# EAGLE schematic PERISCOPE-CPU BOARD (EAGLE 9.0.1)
This Set of Many Schematics Is what comprises the Revision-A PCB, of my eden project "PERISCOPE".

## Sheet 1 of 14: Clock, Horizontal Sync
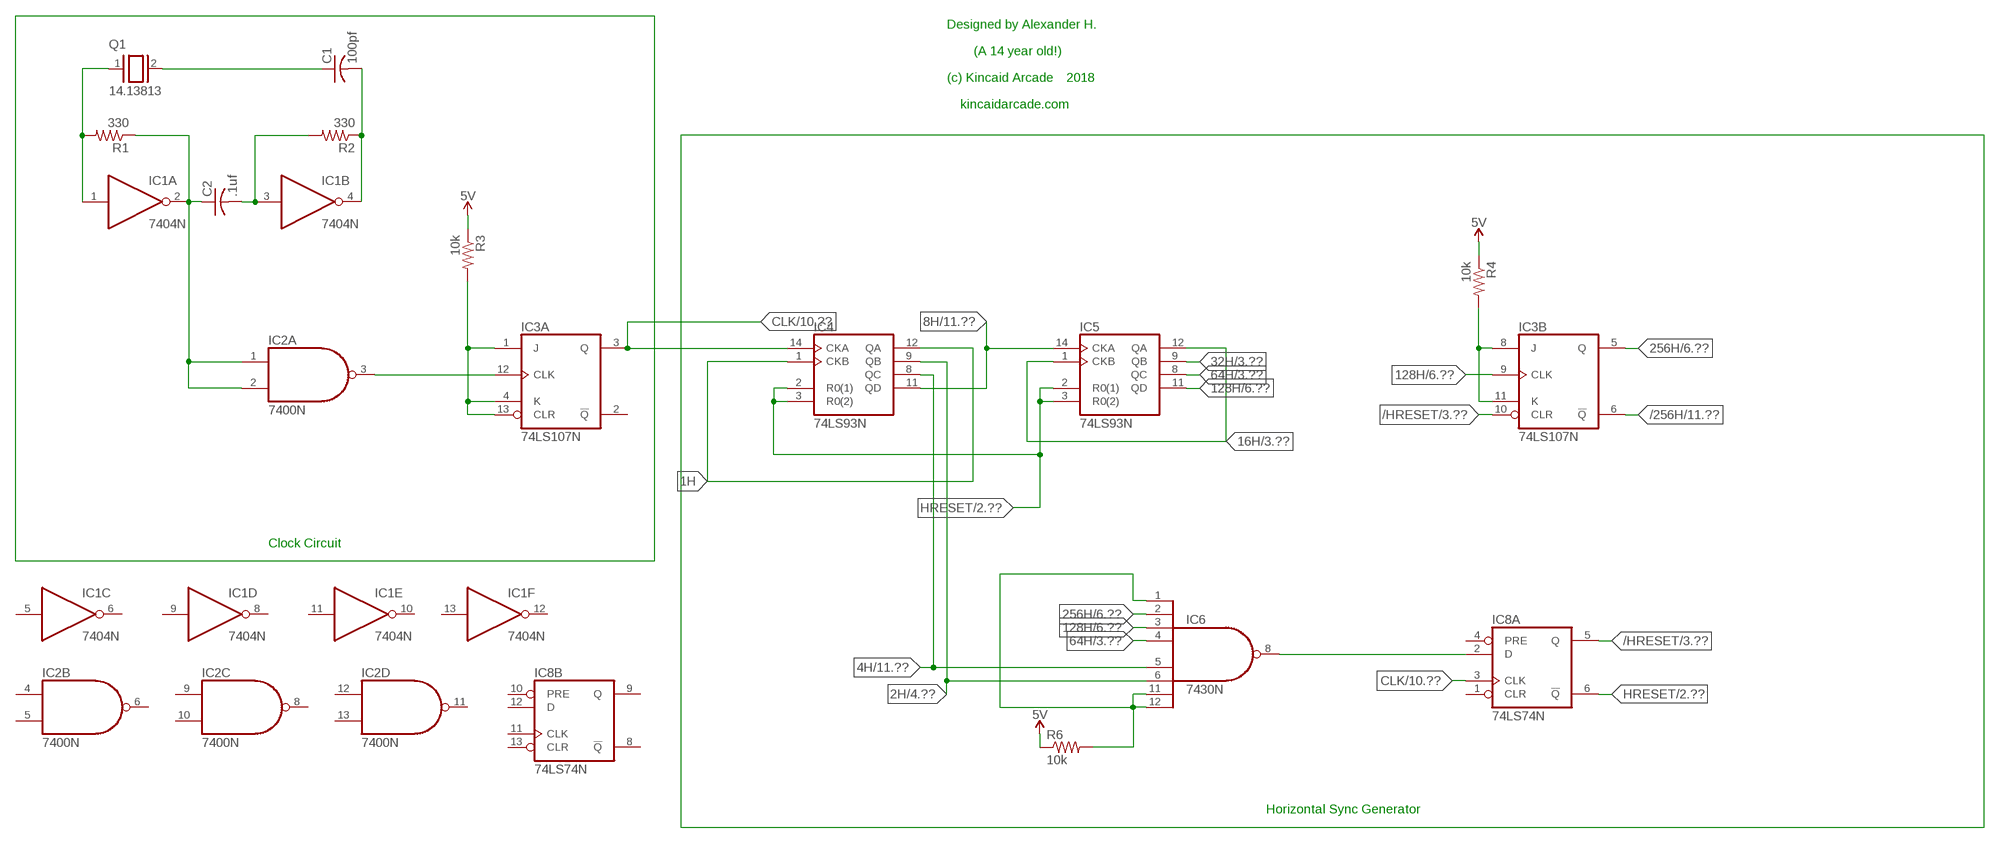
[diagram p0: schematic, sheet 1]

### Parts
C1  100pf  C-US050-025X075  [C050-025X075]
C2  .1uf  C-US050-025X075  [C050-025X075]
IC1  7404N  [DIL14]
IC2  7400N  [DIL14]
IC3  74LS107N  [DIL14]
IC4  74LS93N  [DIL14]
IC5  74LS93N  [DIL14]
IC6  7430N  [DIL14]
IC8  74LS74N  [DIL14]
Q1  14.13813  XTAL/S  [QS]
R1  330  R-US_0207/10  [0207/10]
R2  330  R-US_0207/10  [0207/10]
R3  10k  R-US_0207/10  [0207/10]
R4  10k  R-US_0207/10  [0207/10]
R6  10k  R-US_0207/10  [0207/10]

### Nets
1H: IC4.1(CKB) IC4.12(QA)
2H: IC4.9(QB) IC6.6(I5) ; also sheet 4
4H: IC4.8(QC) IC6.5(I4) ; also sheet 11
5V: R3.1 R4.1 R6.1 ; also sheet 2
8H: IC4.11(QD) IC5.14(CKA) ; also sheet 11
16H: IC5.1(CKB) IC5.12(QA) ; also sheet 3,6,11
32H: IC5.9(QB) ; also sheet 3,6,11
64H: IC5.8(QC) IC6.4(I3) ; also sheet 3,6,11
128H: IC3.9(B:CLK) IC5.11(QD) IC6.3(I2) ; also sheet 6,11
256H: IC3.5(B:Q) IC6.2(I1) ; also sheet 6,11
512H: IC6.1(I0) IC6.11(I6) IC6.12(I7) R6.2
/256H: IC3.6(B:!Q) ; also sheet 11
/HRESET: IC3.10(B:CLR) IC8.5(A:Q) ; also sheet 3
CLK: IC3.3(A:Q) IC4.14(CKA) IC8.3(A:CLK) ; also sheet 10
HRESET: IC4.2(R0(1)) IC4.3(R0(2)) IC5.2(R0(1)) IC5.3(R0(2)) IC8.6(A:!Q) ; also sheet 2,7,8,10
N$1: C1.1 Q1.2
N$2: C1.2 IC1.4(B:O) R2.1
N$3: C2.1 IC1.2(A:O) IC2.1(A:I0) IC2.2(A:I1) R1.1
N$4: C2.2 IC1.3(B:I) R2.2
N$5: IC1.1(A:I) Q1.1 R1.2
N$6: IC2.3(A:O) IC3.12(A:CLK)
N$7: IC3.1(A:J) IC3.4(A:K) IC3.13(A:CLR) R3.2
N$8: IC3.8(B:J) IC3.11(B:K) R4.2
N$11: IC6.8(O) IC8.2(A:D)
Unconnected: IC1.5(C:I) IC1.6(C:O) IC1.8(D:O) IC1.9(D:I) IC1.10(E:O) IC1.11(E:I) IC1.12(F:O) IC1.13(F:I) IC2.4(B:I0) IC2.5(B:I1) IC2.6(B:O) IC2.8(C:O) IC2.9(C:I0) IC2.10(C:I1) IC2.11(D:O) IC2.12(D:I0) IC2.13(D:I1) IC3.2(A:!Q) IC8.1(A:CLR) IC8.4(A:PRE) IC8.8(B:!Q) IC8.9(B:Q) IC8.10(B:PRE) IC8.11(B:CLK) IC8.12(B:D) IC8.13(B:CLR)

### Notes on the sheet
- Designed by Alexander H.
- (A 14 year old!)
- (c) Kincaid Arcade | 2018
- kincaidarcade.com
- Clock Circuit
- Horizontal Sync Generator

## Sheet 2 of 14: Vertical Sync Generator
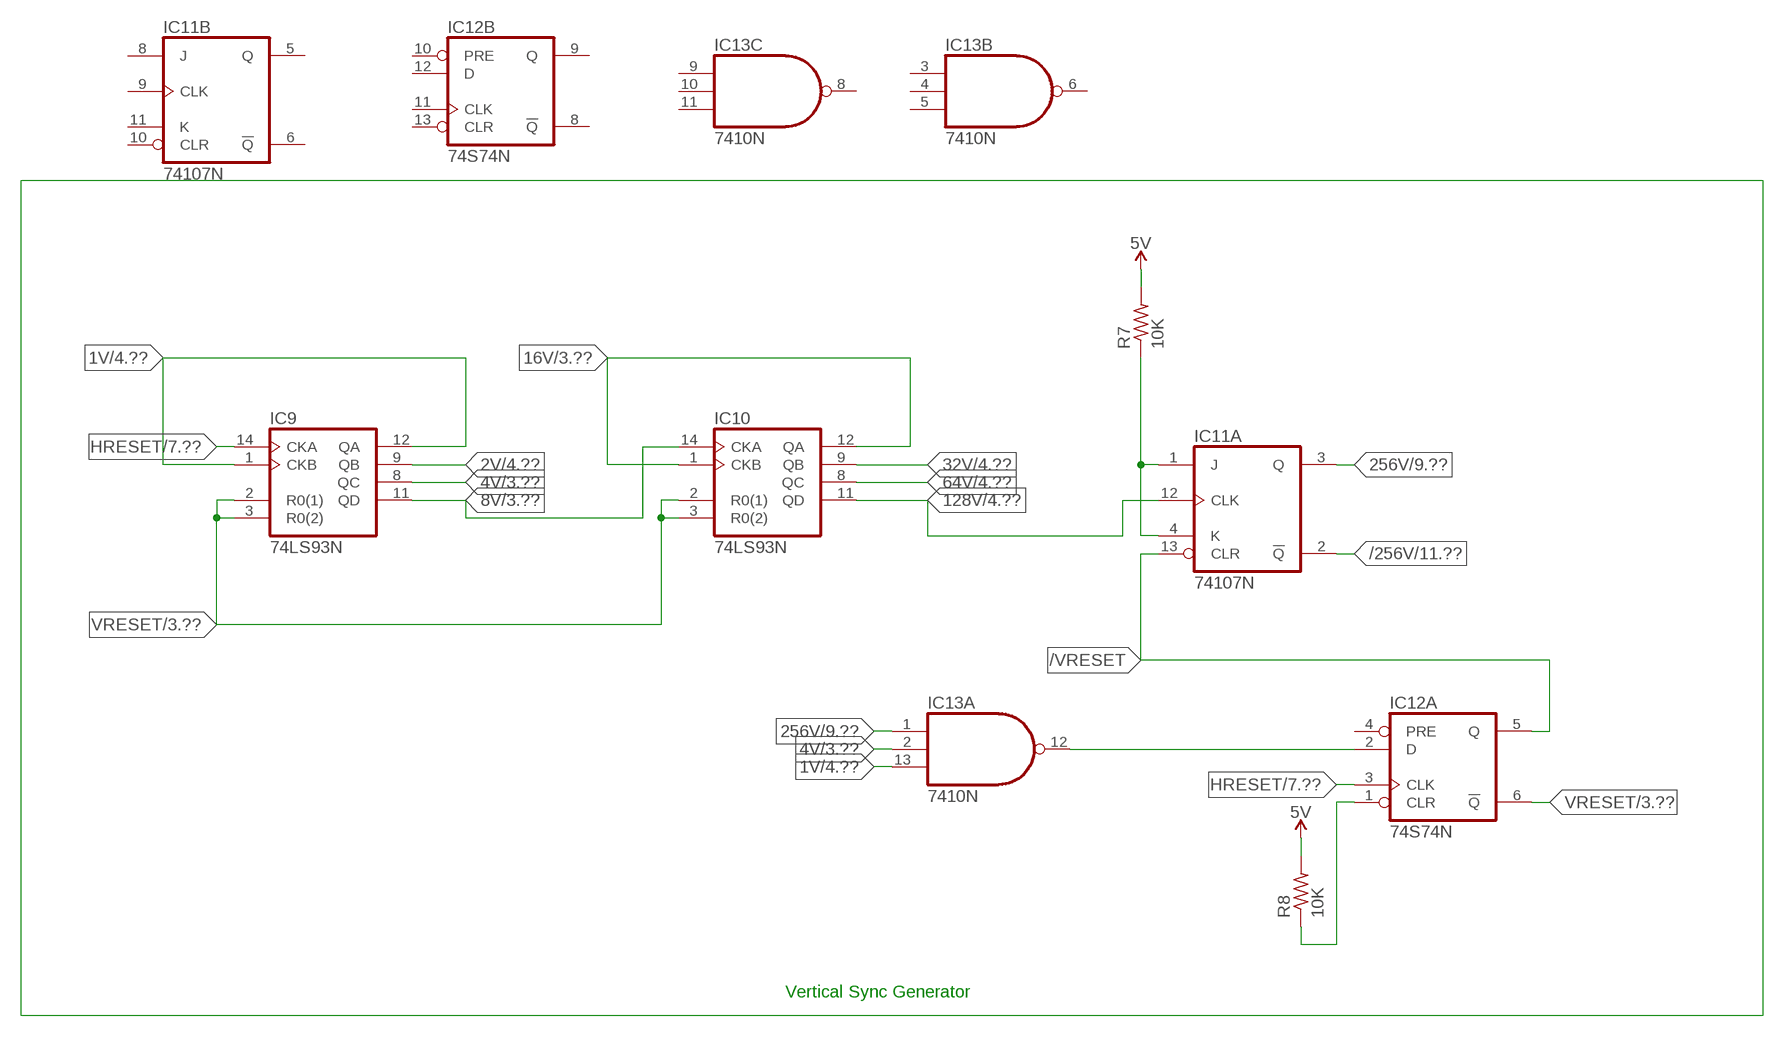
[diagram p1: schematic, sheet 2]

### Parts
IC9  74LS93N  [DIL14]
IC10  74LS93N  [DIL14]
IC11  74107N  [DIL14]
IC12  74S74N  [DIL14]
IC13  7410N  [DIL14]
R7  10K  R-US_0207/10  [0207/10]
R8  10K  R-US_0207/10  [0207/10]

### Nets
1V: IC9.1(CKB) IC9.12(QA) IC13.13(A:I2) ; also sheet 4
2V: IC9.9(QB) ; also sheet 4
4V: IC9.8(QC) IC13.2(A:I1) ; also sheet 3,4,11
5V: R7.2 R8.2 ; also sheet 1
8V: IC9.11(QD) IC10.14(CKA) ; also sheet 3,4,11
16V: IC10.1(CKB) IC10.12(QA) ; also sheet 3,4,5,11
32V: IC10.9(QB) ; also sheet 4,5,11
64V: IC10.8(QC) ; also sheet 4,5
128V: IC10.11(QD) IC11.12(A:CLK) ; also sheet 4,5,9,11
256V: IC11.3(A:Q) IC13.1(A:I0) ; also sheet 9
/256V: IC11.2(A:!Q) ; also sheet 11
/VRESET: IC11.13(A:CLR) IC12.5(A:Q)
HRESET: IC9.14(CKA) IC12.3(A:CLK) ; also sheet 1,7,8,10
N$15: IC11.1(A:J) IC11.4(A:K) R7.1
N$16: IC12.1(A:CLR) R8.1
N$17: IC12.2(A:D) IC13.12(A:O)
VRESET: IC9.2(R0(1)) IC9.3(R0(2)) IC10.2(R0(1)) IC10.3(R0(2)) IC12.6(A:!Q) ; also sheet 3,5
Unconnected: IC11.5(B:Q) IC11.6(B:!Q) IC11.8(B:J) IC11.9(B:CLK) IC11.10(B:CLR) IC11.11(B:K) IC12.4(A:PRE) IC12.8(B:!Q) IC12.9(B:Q) IC12.10(B:PRE) IC12.11(B:CLK) IC12.12(B:D) IC12.13(B:CLR) IC13.3(B:I0) IC13.4(B:I1) IC13.5(B:I2) IC13.6(B:O) IC13.8(C:O) IC13.9(C:I0) IC13.10(C:I1) IC13.11(C:I2)

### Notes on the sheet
- Vertical Sync Generator

## Sheet 3 of 14: Sync Generation
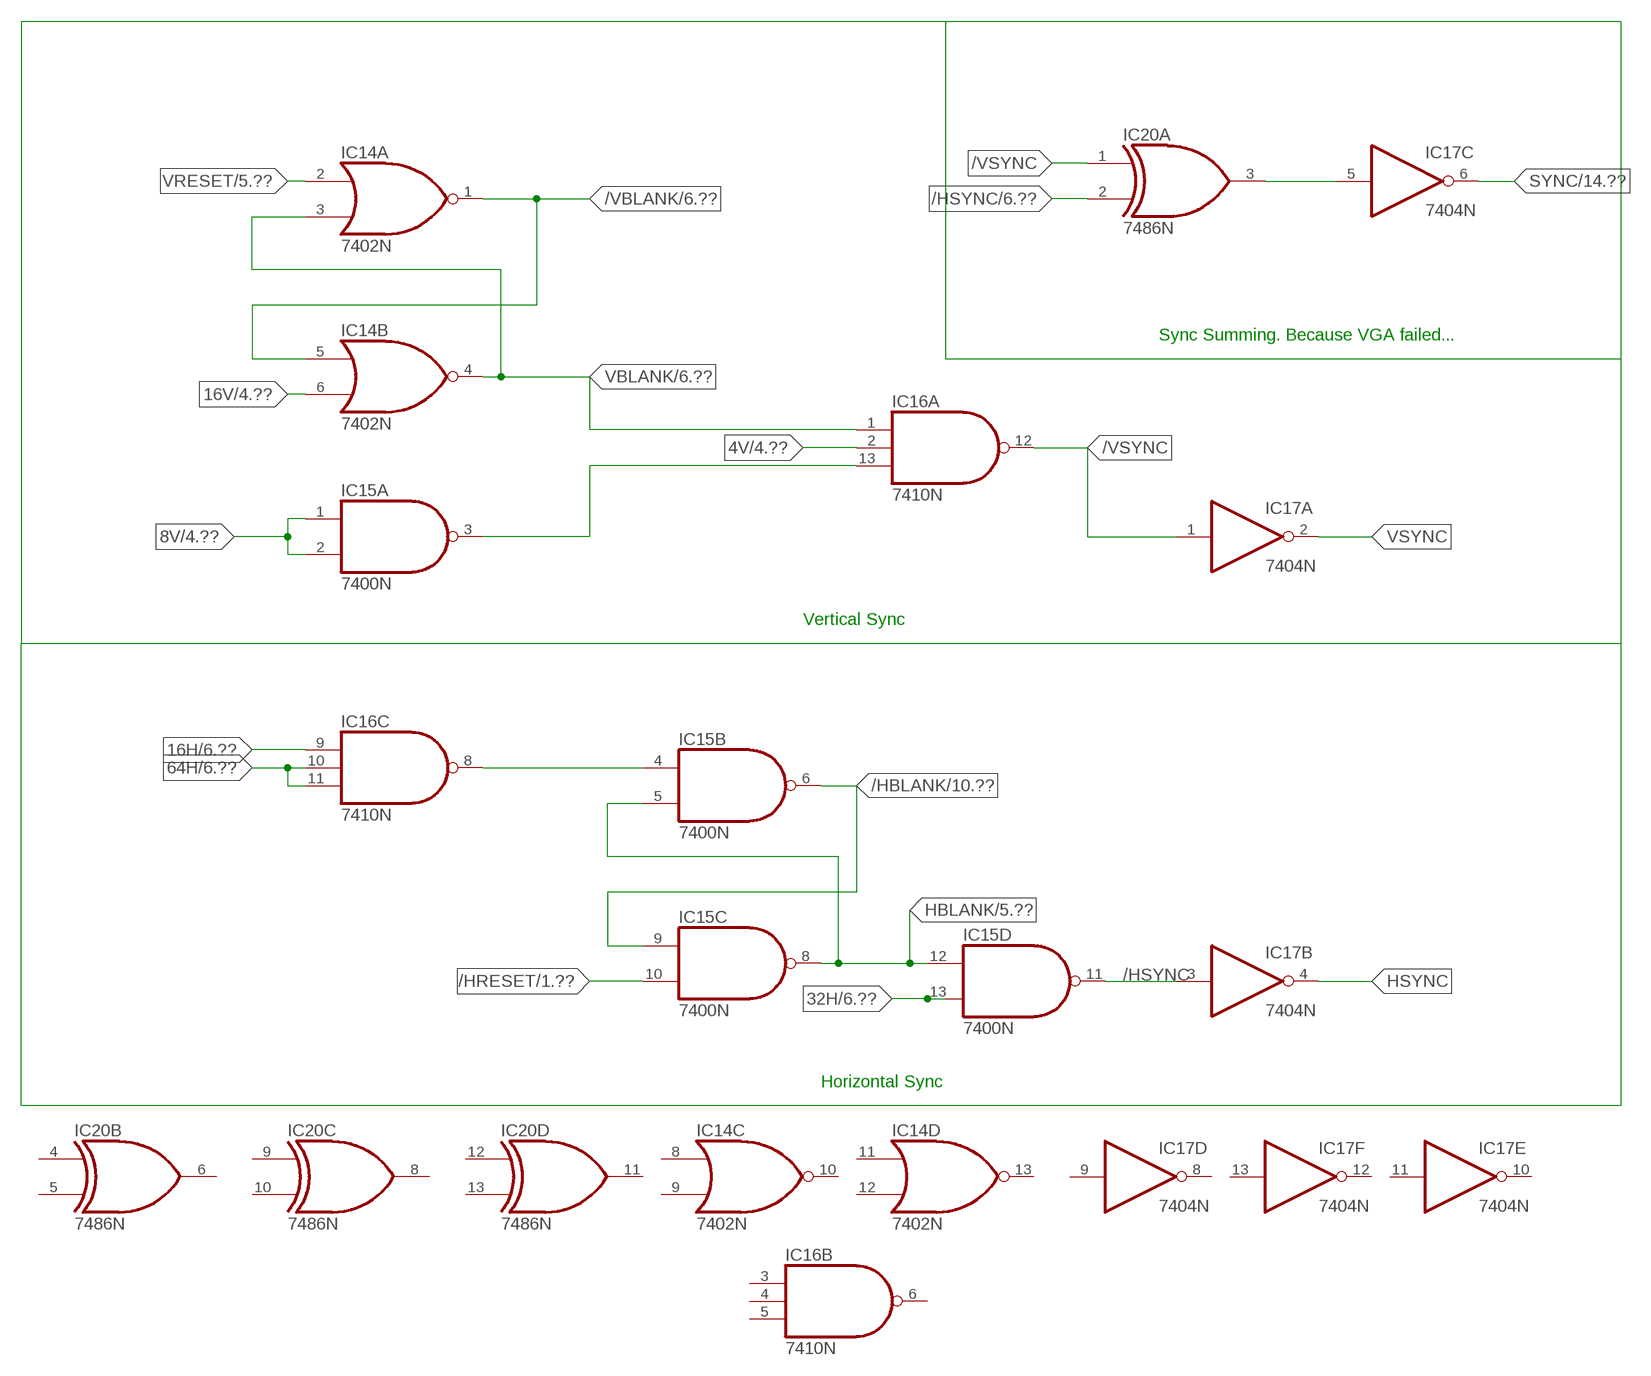
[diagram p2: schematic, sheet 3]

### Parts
IC14  7402N  [DIL14]
IC15  7400N  [DIL14]
IC16  7410N  [DIL14]
IC17  7404N  [DIL14]
IC20  7486N  [DIL14]

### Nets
4V: IC16.2(A:I1) ; also sheet 2,4,11
8V: IC15.1(A:I0) IC15.2(A:I1) ; also sheet 2,4,11
16H: IC16.9(C:I0) ; also sheet 1,6,11
16V: IC14.6(B:I1) ; also sheet 2,4,5,11
32H: IC15.13(D:I1) ; also sheet 1,6,11
64H: IC16.10(C:I1) IC16.11(C:I2) ; also sheet 1,6,11
/HBLANK: IC15.6(B:O) IC15.9(C:I0) ; also sheet 10
/HRESET: IC15.10(C:I1) ; also sheet 1
/HSYNC: IC15.11(D:O) IC17.3(B:I) IC20.2(A:I1) ; also sheet 6,10
/VBLANK: IC14.1(A:O) IC14.5(B:I0) ; also sheet 6,10
/VSYNC: IC16.12(A:O) IC17.1(A:I) IC20.1(A:I0)
HBLANK: IC15.5(B:I1) IC15.8(C:O) IC15.12(D:I0) ; also sheet 5,10
HSYNC: IC17.4(B:O)
N$19: IC15.4(B:I0) IC16.8(C:O)
N$20: IC15.3(A:O) IC16.13(A:I2)
N$22: IC17.5(C:I) IC20.3(A:O)
SYNC: IC17.6(C:O) ; also sheet 14
VBLANK: IC14.3(A:I1) IC14.4(B:O) IC16.1(A:I0) ; also sheet 6
VRESET: IC14.2(A:I0) ; also sheet 2,5
VSYNC: IC17.2(A:O)
Unconnected: IC14.8(C:I0) IC14.9(C:I1) IC14.10(C:O) IC14.11(D:I0) IC14.12(D:I1) IC14.13(D:O) IC16.3(B:I0) IC16.4(B:I1) IC16.5(B:I2) IC16.6(B:O) IC17.8(D:O) IC17.9(D:I) IC17.10(E:O) IC17.11(E:I) IC17.12(F:O) IC17.13(F:I) IC20.4(B:I0) IC20.5(B:I1) IC20.6(B:O) IC20.8(C:O) IC20.9(C:I0) IC20.10(C:I1) IC20.11(D:O) IC20.12(D:I0) IC20.13(D:I1)

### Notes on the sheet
- Sync Summing. Because VGA failed...
- Vertical Sync
- Horizontal Sync

## Sheet 4 of 14: Ocean Generation, Surface and Floor
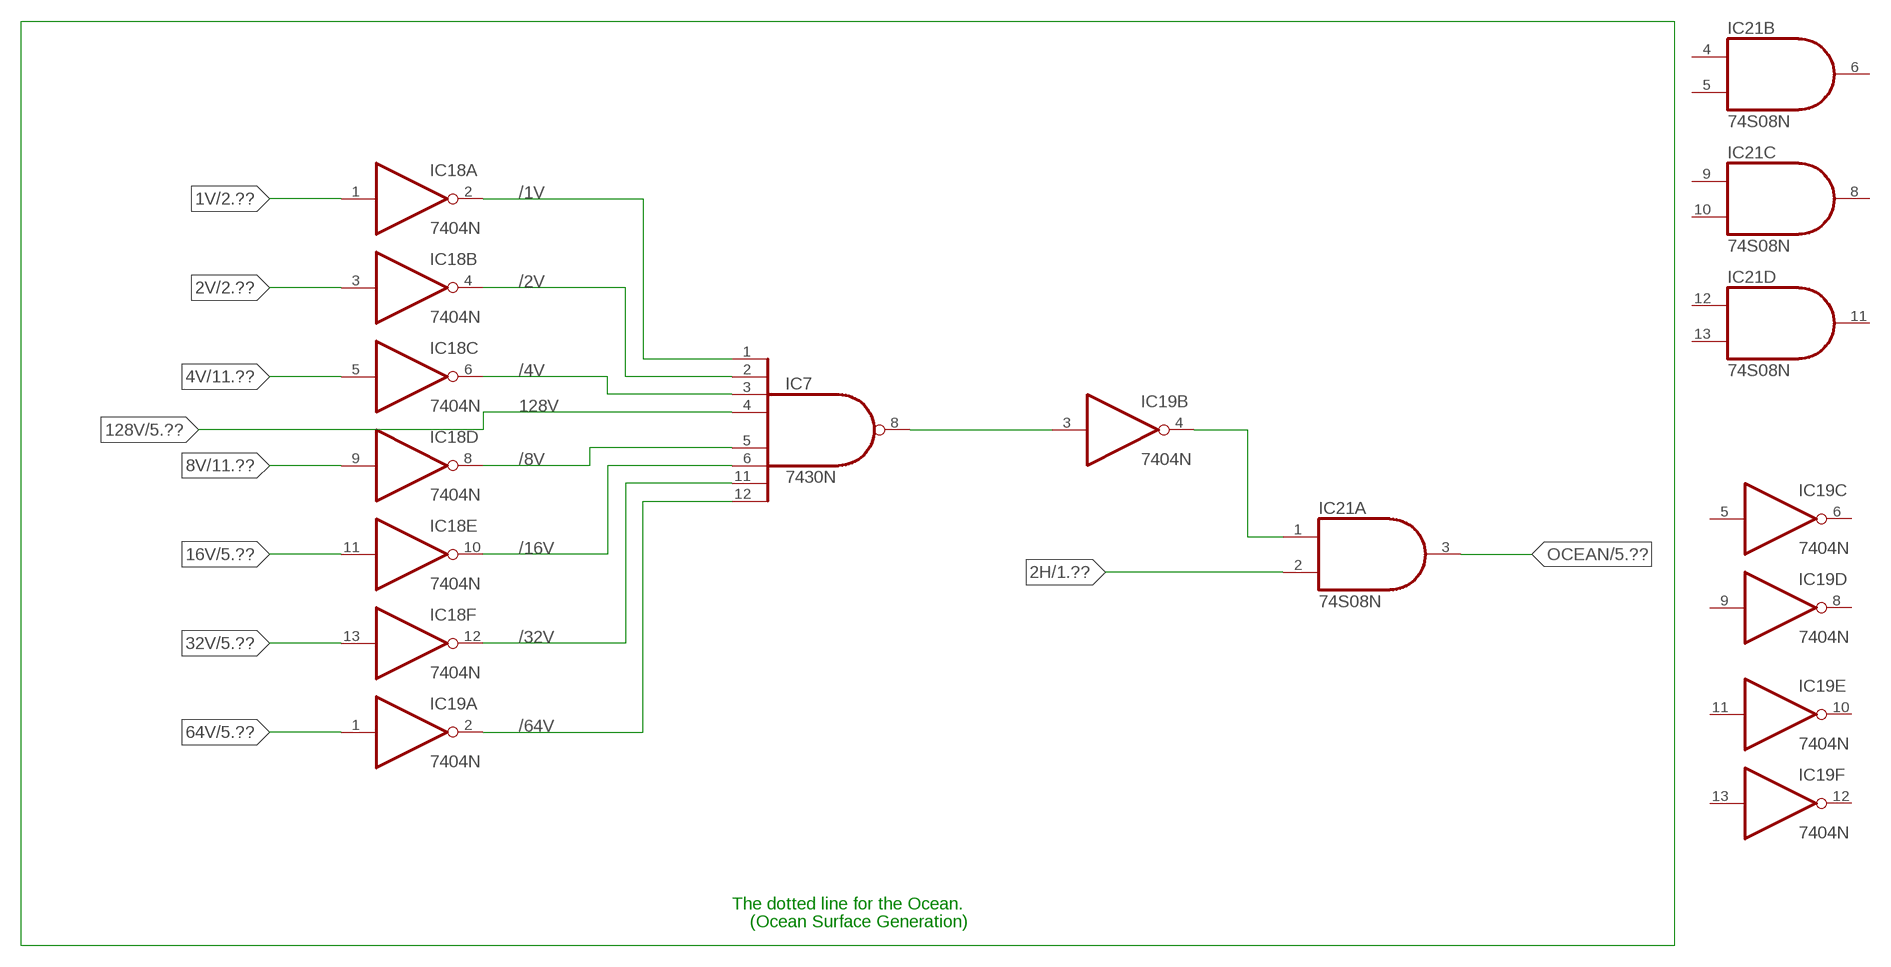
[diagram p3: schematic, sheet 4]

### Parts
IC7  7430N  [DIL14]
IC18  7404N  [DIL14]
IC19  7404N  [DIL14]
IC21  74S08N  [DIL14]

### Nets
1V: IC18.1(A:I) ; also sheet 2
2H: IC21.2(A:I1) ; also sheet 1
2V: IC18.3(B:I) ; also sheet 2
4V: IC18.5(C:I) ; also sheet 2,3,11
8V: IC18.9(D:I) ; also sheet 2,3,11
16V: IC18.11(E:I) ; also sheet 2,3,5,11
32V: IC18.13(F:I) ; also sheet 2,5,11
64V: IC19.1(A:I) ; also sheet 2,5
128V: IC7.4(I3) ; also sheet 2,5,9,11
/1V: IC7.1(I0) IC18.2(A:O)
/2V: IC7.2(I1) IC18.4(B:O)
/4V: IC7.3(I2) IC18.6(C:O)
/8V: IC7.5(I4) IC18.8(D:O)
/16V: IC7.6(I5) IC18.10(E:O)
/32V: IC7.11(I6) IC18.12(F:O)
/64V: IC7.12(I7) IC19.2(A:O) ; also sheet 11
N$28: IC7.8(O) IC19.3(B:I)
N$29: IC19.4(B:O) IC21.1(A:I0)
OCEAN: IC21.3(A:O) ; also sheet 5,6,10,13
Unconnected: IC19.5(C:I) IC19.6(C:O) IC19.8(D:O) IC19.9(D:I) IC19.10(E:O) IC19.11(E:I) IC19.12(F:O) IC19.13(F:I) IC21.4(B:I0) IC21.5(B:I1) IC21.6(B:O) IC21.8(C:O) IC21.9(C:I0) IC21.10(C:I1) IC21.11(D:O) IC21.12(D:I0) IC21.13(D:I1)

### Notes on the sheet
- The dotted line for the Ocean.
- (Ocean Surface Generation)

## Sheet 5 of 14: Freighter Generation
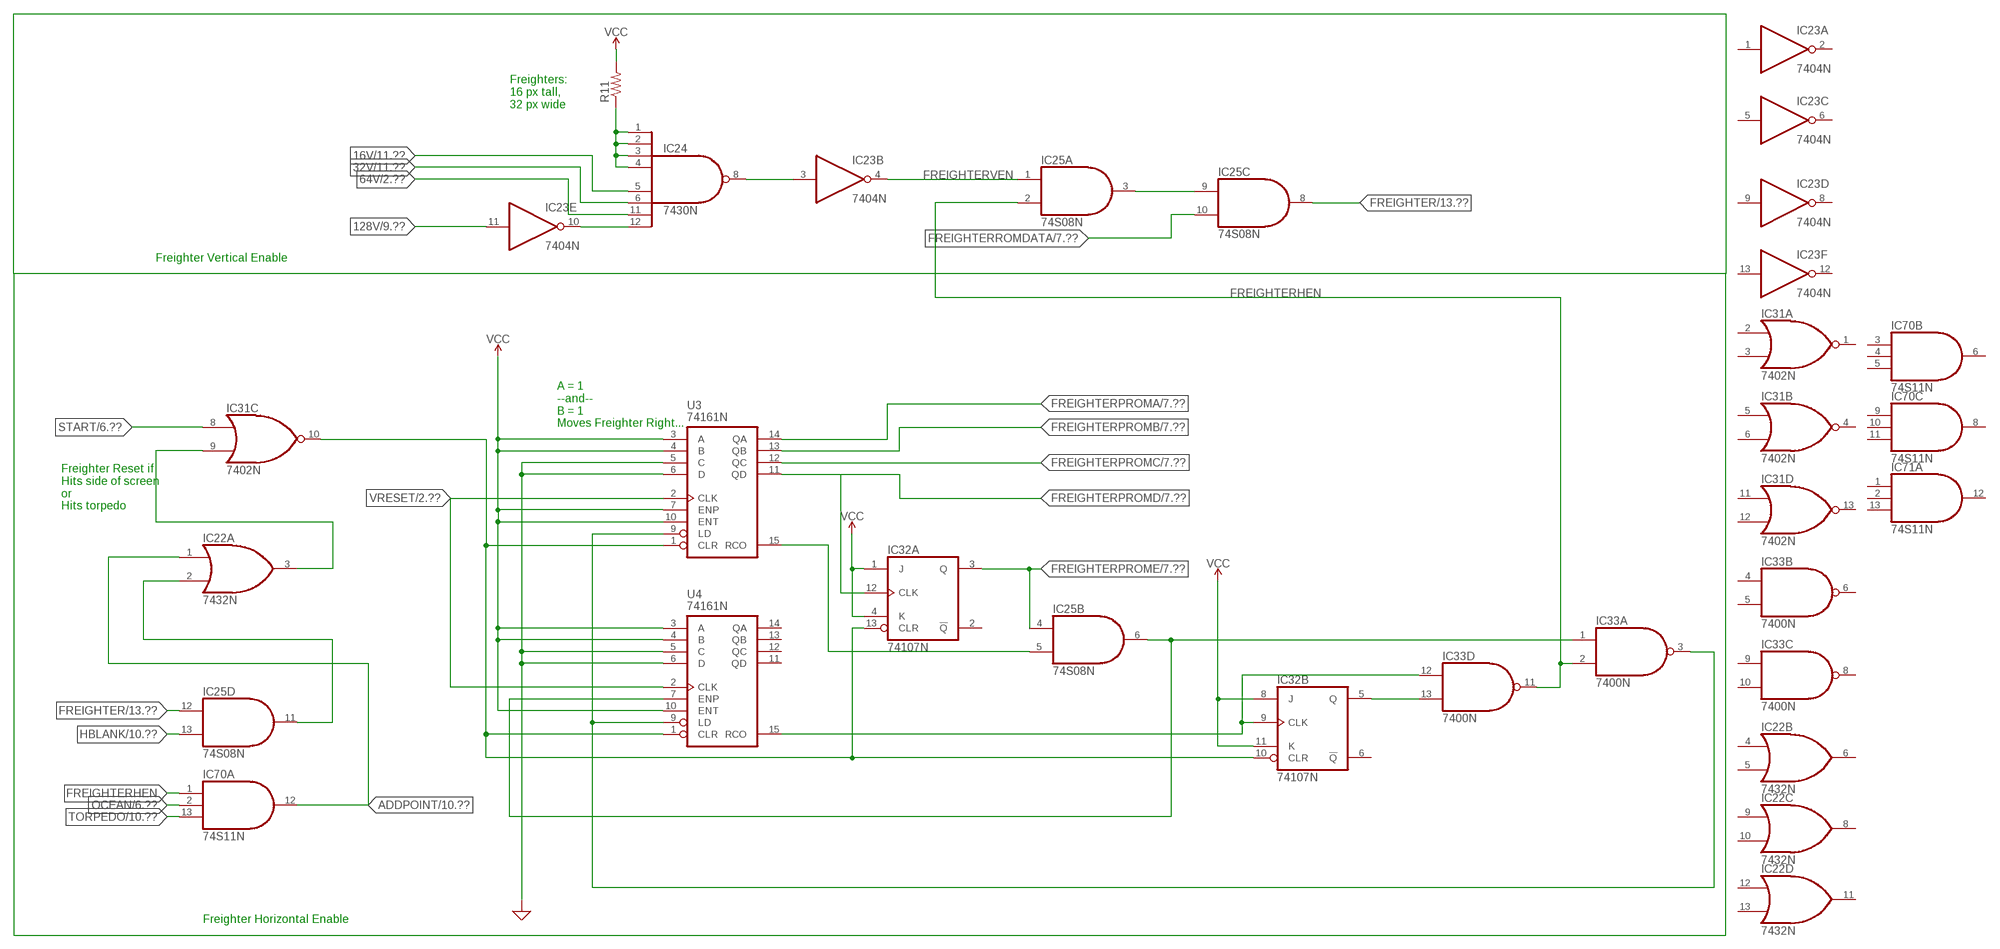
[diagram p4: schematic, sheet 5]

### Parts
IC22  7432N  [DIL14]
IC23  7404N  [DIL14]
IC24  7430N  [DIL14]
IC25  74S08N  [DIL14]
IC31  7402N  [DIL14]
IC32  74107N  [DIL14]
IC33  7400N  [DIL14]
IC70  74S11N  [DIL14]
IC71  74S11N  [DIL14]
R11  R-US_0207/10  [0207/10]
U3  74161N  [DIL16]
U4  74161N  [DIL16]

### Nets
16V: IC24.5(I4) ; also sheet 2,3,4,11
32V: IC24.6(I5) ; also sheet 2,4,11
64V: IC24.11(I6) ; also sheet 2,4
128V: IC23.11(E:I) ; also sheet 2,4,9,11
ADDPOINT: IC22.1(A:I0) IC70.12(A:O) ; also sheet 10,11
FREIGHTER: IC25.8(C:O) IC25.12(D:I0) ; also sheet 13
FREIGHTERHEN: IC25.2(A:I1) IC33.2(A:I1) IC33.11(D:O) IC70.1(A:I0)
FREIGHTERPROMA: U3.14(QA) ; also sheet 7
FREIGHTERPROMB: U3.13(QB) ; also sheet 7
FREIGHTERPROMC: U3.12(QC) ; also sheet 7
FREIGHTERPROMD: IC32.12(A:CLK) U3.11(QD) ; also sheet 7
FREIGHTERPROME: IC25.4(B:I0) IC32.3(A:Q) ; also sheet 7
FREIGHTERROMDATA: IC25.10(C:I1) ; also sheet 7
FREIGHTERVEN: IC23.4(B:O) IC25.1(A:I0) ; also sheet 7
GND: U3.5(C) U3.6(D) U4.5(C) U4.6(D) ; supply symbol labelled SUP ; also sheet 6,7,8,9,10,11,14
HBLANK: IC22.3(A:O) IC25.13(D:I1) IC31.9(C:I1) ; also sheet 3,10
N$21: IC31.10(C:O) IC32.10(B:CLR) IC32.13(A:CLR) U3.1(CLR) U4.1(CLR)
N$24: IC25.5(B:I1) U3.15(RCO)
N$25: IC25.6(B:O) IC33.1(A:I0) U4.7(ENP)
N$27: IC32.5(B:Q) IC33.13(D:I1)
N$31: IC22.2(A:I1) IC25.11(D:O)
N$35: IC23.10(E:O) IC24.12(I7)
N$36: IC23.3(B:I) IC24.8(O)
N$37: IC25.3(A:O) IC25.9(C:I0)
N$40: IC24.1(I0) IC24.2(I1) IC24.3(I2) IC24.4(I3) R11.1
N$53: IC32.9(B:CLK) IC33.12(D:I0) U4.15(RCO)
N$54: IC33.3(A:O) U3.9(LD) U4.9(LD)
OCEAN: IC70.2(A:I1) ; also sheet 4,6,10,13
START: IC31.8(C:I0) ; also sheet 6,9,11
TORPEDO: IC70.13(A:I2) ; also sheet 10,13
VCC: IC32.1(A:J) IC32.4(A:K) IC32.8(B:J) IC32.11(B:K) R11.2 U3.3(A) U3.4(B) U3.7(ENP) U3.10(ENT) U4.3(A) U4.4(B) U4.10(ENT) ; also sheet 6,7,8,9,10,11,14
VRESET: U3.2(CLK) U4.2(CLK) ; also sheet 2,3
Unconnected: IC22.4(B:I0) IC22.5(B:I1) IC22.6(B:O) IC22.8(C:O) IC22.9(C:I0) IC22.10(C:I1) IC22.11(D:O) IC22.12(D:I0) IC22.13(D:I1) IC23.1(A:I) IC23.2(A:O) IC23.5(C:I) IC23.6(C:O) IC23.8(D:O) IC23.9(D:I) IC23.12(F:O) IC23.13(F:I) IC31.1(A:O) IC31.2(A:I0) IC31.3(A:I1) IC31.4(B:O) IC31.5(B:I0) IC31.6(B:I1) IC31.11(D:I0) IC31.12(D:I1) IC31.13(D:O) IC32.2(A:!Q) IC32.6(B:!Q) IC33.4(B:I0) IC33.5(B:I1) IC33.6(B:O) IC33.8(C:O) IC33.9(C:I0) IC33.10(C:I1) IC70.3(B:I0) IC70.4(B:I1) IC70.5(B:I2) IC70.6(B:O) IC70.8(C:O) IC70.9(C:I0) IC70.10(C:I1) IC70.11(C:I2) IC71.1(A:I0) IC71.2(A:I1) IC71.3(B:I0) IC71.4(B:I1) IC71.5(B:I2) IC71.6(B:O) IC71.8(C:O) IC71.9(C:I0) IC71.10(C:I1) IC71.11(C:I2) IC71.12(A:O) IC71.13(A:I2) U4.11(QD) U4.12(QC) U4.13(QB) U4.14(QA)

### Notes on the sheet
- Freighters:
  16 px tall,
  32 px wide
- Freighter Vertical Enable
- A = 1 
  --and--
  B = 1
  Moves Freighter Right...
- Freighter Reset if 
  Hits side of screen
  or
  Hits torpedo
- Freighter Horizontal Enable

## Sheet 6 of 14: Submarine Generation
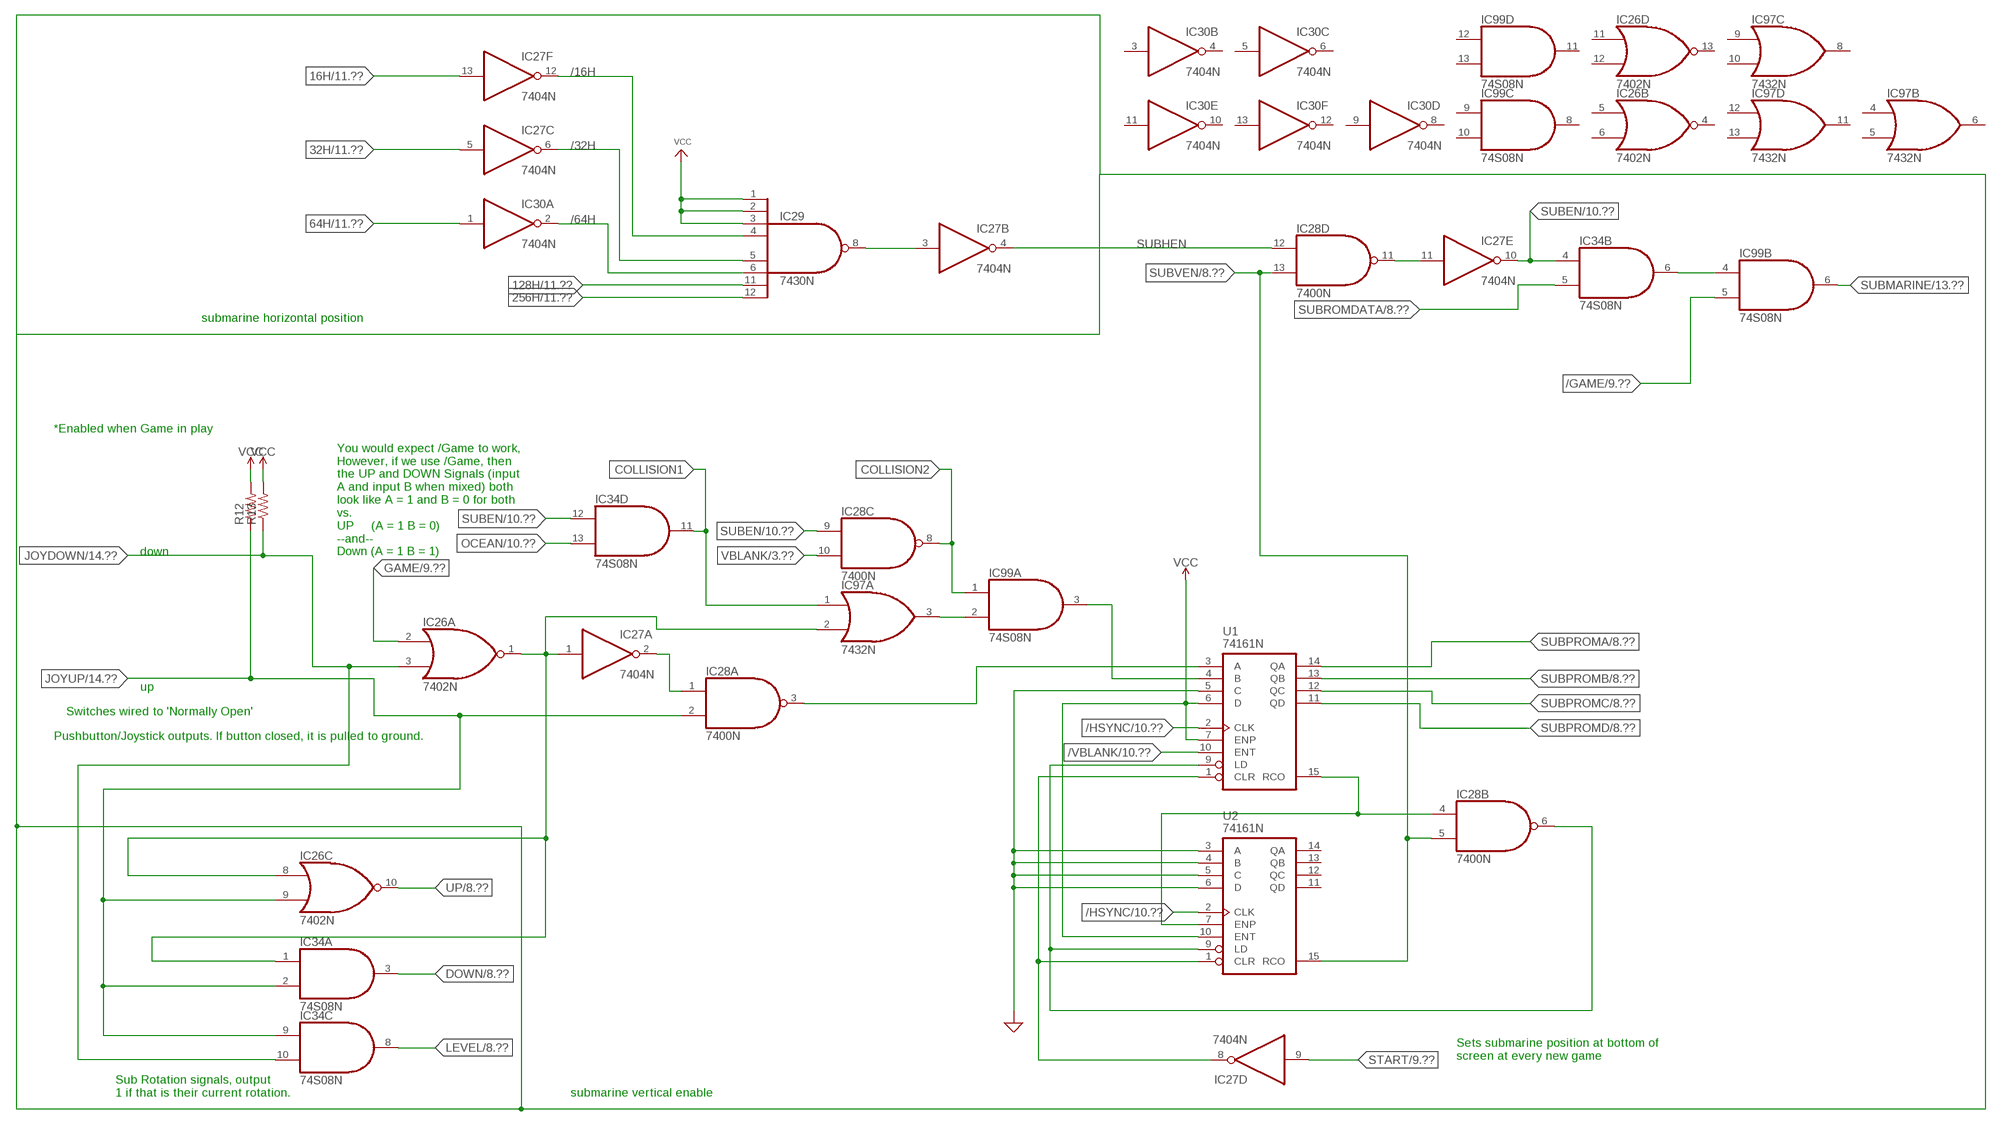
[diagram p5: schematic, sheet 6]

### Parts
IC26  7402N  [DIL14]
IC27  7404N  [DIL14]
IC28  7400N  [DIL14]
IC29  7430N  [DIL14]
IC30  7404N  [DIL14]
IC34  74S08N  [DIL14]
IC97  7432N  [DIL14]
IC99  74S08N  [DIL14]
R12  R-US_0207/10  [0207/10]
R13  R-US_0207/10  [0207/10]
U1  74161N  [DIL16]
U2  74161N  [DIL16]

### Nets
16H: IC27.13(F:I) ; also sheet 1,3,11
32H: IC27.5(C:I) ; also sheet 1,3,11
64H: IC30.1(A:I) ; also sheet 1,3,11
128H: IC29.11(I6) ; also sheet 1,11
256H: IC29.12(I7) ; also sheet 1,11
/16H: IC27.12(F:O) IC29.4(I3)
/32H: IC27.6(C:O) IC29.5(I4) ; also sheet 11
/64H: IC29.6(I5) IC30.2(A:O) ; also sheet 11
/GAME: IC99.5(B:I1) ; also sheet 9,10
/HSYNC: U1.2(CLK) U2.2(CLK) ; also sheet 3,10
/VBLANK: U1.10(ENT) ; also sheet 3,10
COLLISION1: IC34.11(D:O) IC97.1(A:I0)
COLLISION2: IC28.8(C:O) IC99.1(A:I0)
DOWN: IC34.3(A:O) ; also sheet 8,10
GAME: IC26.2(A:I0) ; also sheet 9
GND: U1.5(C) U2.3(A) U2.4(B) U2.5(C) U2.6(D) ; supply symbol labelled SUP ; also sheet 5,7,8,9,10,11,14
GSTART: IC27.8(D:O) U1.1(CLR) U2.1(CLR)
JOYDOWN: IC26.3(A:I1) IC34.10(C:I1) R13.1 ; also sheet 14
JOYUP: IC26.9(C:I1) IC28.2(A:I1) IC34.2(A:I1) IC34.9(C:I0) R12.1 ; also sheet 14
LEVEL: IC34.8(C:O) ; also sheet 8
N$42: IC27.2(A:O) IC28.1(A:I0)
N$43: IC26.1(A:O) IC26.8(C:I0) IC27.1(A:I) IC34.1(A:I0) IC97.2(A:I1)
N$44: IC28.4(B:I0) U1.15(RCO) U2.7(ENP)
N$45: IC27.3(B:I) IC29.8(O)
N$46: IC28.6(B:O) U1.9(LD) U2.9(LD)
N$47: IC27.11(E:I) IC28.11(D:O)
N$48: IC97.3(A:O) IC99.2(A:I1)
N$186: IC99.3(A:O) U1.4(B)
N$190: IC28.3(A:O) U1.3(A)
N$210: IC34.6(B:O) IC99.4(B:I0)
OCEAN: IC34.13(D:I1) ; also sheet 4,5,10,13
START: IC27.9(D:I) ; also sheet 5,9,11
SUBEN: IC27.10(E:O) IC28.9(C:I0) IC34.4(B:I0) IC34.12(D:I0) ; also sheet 10
SUBHEN: IC27.4(B:O) IC28.12(D:I0) ; also sheet 10
SUBMARINE: IC99.6(B:O) ; also sheet 13
SUBPROMA: U1.14(QA) ; also sheet 8,10
SUBPROMB: U1.13(QB) ; also sheet 8,10
SUBPROMC: U1.12(QC) ; also sheet 8,10
SUBPROMD: U1.11(QD) ; also sheet 8,10
SUBROMDATA: IC34.5(B:I1) ; also sheet 8
SUBVEN: IC28.5(B:I1) IC28.13(D:I1) U2.15(RCO) ; also sheet 8,10
UP: IC26.10(C:O) ; also sheet 8,10
VBLANK: IC28.10(C:I1) ; also sheet 3
VCC: IC29.1(I0) IC29.2(I1) IC29.3(I2) R12.2 R13.2 U1.6(D) U1.7(ENP) U2.10(ENT) ; also sheet 5,7,8,9,10,11,14
Unconnected: IC26.4(B:O) IC26.5(B:I0) IC26.6(B:I1) IC26.11(D:I0) IC26.12(D:I1) IC26.13(D:O) IC30.3(B:I) IC30.4(B:O) IC30.5(C:I) IC30.6(C:O) IC30.8(D:O) IC30.9(D:I) IC30.10(E:O) IC30.11(E:I) IC30.12(F:O) IC30.13(F:I) IC97.4(B:I0) IC97.5(B:I1) IC97.6(B:O) IC97.8(C:O) IC97.9(C:I0) IC97.10(C:I1) IC97.11(D:O) IC97.12(D:I0) IC97.13(D:I1) IC99.8(C:O) IC99.9(C:I0) IC99.10(C:I1) IC99.11(D:O) IC99.12(D:I0) IC99.13(D:I1) U2.11(QD) U2.12(QC) U2.13(QB) U2.14(QA)

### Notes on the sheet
- submarine horizontal position
- *Enabled when Game in play
- down
- You would expect /Game to work,
  However, if we use /Game, then 
  the UP and DOWN Signals (input
  A and input B when mixed) both
  look like A = 1 and B = 0 for both
  vs. 
  UP     (A = 1 B = 0)
  --and--
  Down (A = 1 B = 1)
- up
- Switches wired to 'Normally Open'
- Pushbutton/Joystick outputs. If button closed, it is pulled to ground.
- Sets submarine position at bottom of
  screen at every new game
- Sub Rotation signals, output
  1 if that is their current rotation.
- submarine vertical enable

## Sheet 7 of 14: Freighter Prom data/addressing
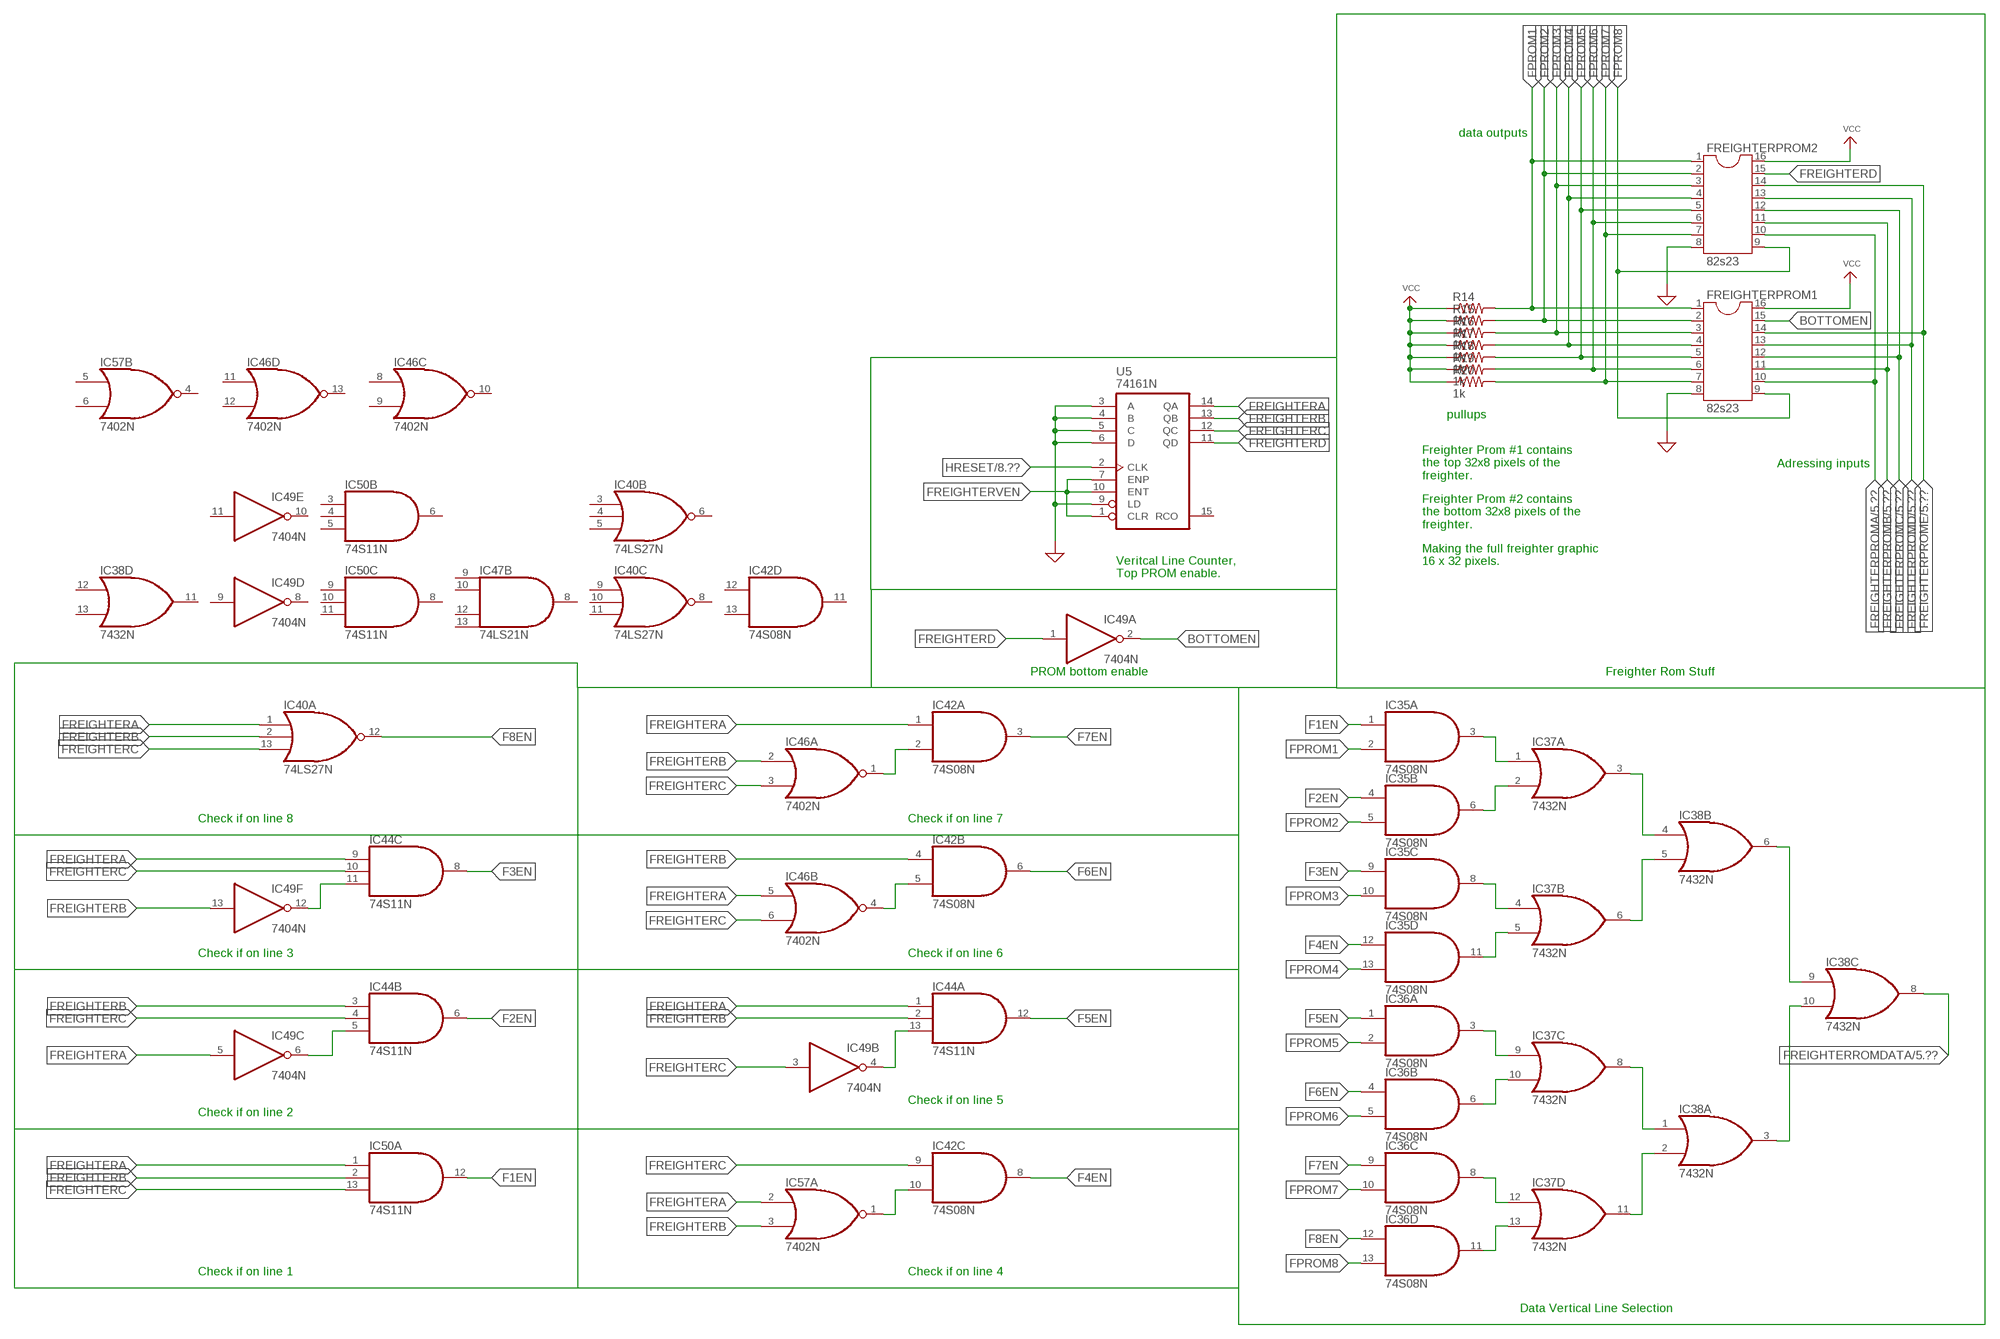
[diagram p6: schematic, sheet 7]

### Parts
FREIGHTERPROM1  82s23  DIL16  [DIL16]
FREIGHTERPROM2  82s23  DIL16  [DIL16]
IC35  74S08N  [DIL14]
IC36  74S08N  [DIL14]
IC37  7432N  [DIL14]
IC38  7432N  [DIL14]
IC40  74LS27N  [DIL14]
IC42  74S08N  [DIL14]
IC44  74S11N  [DIL14]
IC46  7402N  [DIL14]
IC47  74LS21N  [DIL14]
IC49  7404N  [DIL14]
IC50  74S11N  [DIL14]
IC57  7402N  [DIL14]
R14  1k  R-US_0207/10  [0207/10]
R15  1k  R-US_0207/10  [0207/10]
R16  1k  R-US_0207/10  [0207/10]
R17  1k  R-US_0207/10  [0207/10]
R18  1k  R-US_0207/10  [0207/10]
R19  1k  R-US_0207/10  [0207/10]
R20  1k  R-US_0207/10  [0207/10]
U5  74161N  [DIL16]

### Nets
BOTTOMEN: FREIGHTERPROM1.15 IC49.2(A:O)
F1EN: IC35.1(A:I0) IC50.12(A:O)
F2EN: IC35.4(B:I0) IC44.6(B:O)
F3EN: IC35.9(C:I0) IC44.8(C:O)
F4EN: IC35.12(D:I0) IC42.8(C:O)
F5EN: IC36.1(A:I0) IC44.12(A:O)
F6EN: IC36.4(B:I0) IC42.6(B:O)
F7EN: IC36.9(C:I0) IC42.3(A:O)
F8EN: IC36.12(D:I0) IC40.12(A:O)
FPROM1: FREIGHTERPROM1.1 FREIGHTERPROM2.1 IC35.2(A:I1) R14.2
FPROM2: FREIGHTERPROM1.2 FREIGHTERPROM2.2 IC35.5(B:I1) R15.2
FPROM3: FREIGHTERPROM1.3 FREIGHTERPROM2.3 IC35.10(C:I1) R16.2
FPROM4: FREIGHTERPROM1.4 FREIGHTERPROM2.4 IC35.13(D:I1) R17.2
FPROM5: FREIGHTERPROM1.5 FREIGHTERPROM2.5 IC36.2(A:I1) R18.2
FPROM6: FREIGHTERPROM1.6 FREIGHTERPROM2.6 IC36.5(B:I1) R19.2
FPROM7: FREIGHTERPROM1.7 FREIGHTERPROM2.7 IC36.10(C:I1) R20.2
FPROM8: FREIGHTERPROM1.9 FREIGHTERPROM2.9 IC36.13(D:I1)
FREIGHTERA: IC40.1(A:I0) IC42.1(A:I0) IC44.1(A:I0) IC44.9(C:I0) IC46.5(B:I0) IC49.5(C:I) IC50.1(A:I0) IC57.2(A:I0) U5.14(QA)
FREIGHTERB: IC40.2(A:I1) IC42.4(B:I0) IC44.2(A:I1) IC44.3(B:I0) IC46.2(A:I0) IC49.13(F:I) IC50.2(A:I1) IC57.3(A:I1) U5.13(QB)
FREIGHTERC: IC40.13(A:I2) IC42.9(C:I0) IC44.4(B:I1) IC44.10(C:I1) IC46.3(A:I1) IC46.6(B:I1) IC49.3(B:I) IC50.13(A:I2) U5.12(QC)
FREIGHTERD: FREIGHTERPROM2.15 IC49.1(A:I) U5.11(QD)
FREIGHTERPROMA: FREIGHTERPROM1.10 FREIGHTERPROM2.10 ; also sheet 5
FREIGHTERPROMB: FREIGHTERPROM1.11 FREIGHTERPROM2.11 ; also sheet 5
FREIGHTERPROMC: FREIGHTERPROM1.12 FREIGHTERPROM2.12 ; also sheet 5
FREIGHTERPROMD: FREIGHTERPROM1.13 FREIGHTERPROM2.13 ; also sheet 5
FREIGHTERPROME: FREIGHTERPROM1.14 FREIGHTERPROM2.14 ; also sheet 5
FREIGHTERROMDATA: IC38.8(C:O) ; also sheet 5
FREIGHTERVEN: U5.1(CLR) U5.7(ENP) U5.10(ENT) ; also sheet 5
GND: FREIGHTERPROM1.8 FREIGHTERPROM2.8 U5.3(A) U5.4(B) U5.5(C) U5.6(D) U5.9(LD) ; supply symbol labelled SUP ; also sheet 5,6,8,9,10,11,14
HRESET: U5.2(CLK) ; also sheet 1,2,8,10
N$41: IC35.6(B:O) IC37.2(A:I1)
N$51: IC35.3(A:O) IC37.1(A:I0)
N$52: IC35.8(C:O) IC37.4(B:I0)
N$55: IC35.11(D:O) IC37.5(B:I1)
N$56: IC36.3(A:O) IC37.9(C:I0)
N$57: IC36.6(B:O) IC37.10(C:I1)
N$58: IC36.8(C:O) IC37.12(D:I0)
N$59: IC36.11(D:O) IC37.13(D:I1)
N$60: IC37.11(D:O) IC38.2(A:I1)
N$61: IC37.8(C:O) IC38.1(A:I0)
N$62: IC37.6(B:O) IC38.5(B:I1)
N$63: IC37.3(A:O) IC38.4(B:I0)
N$64: IC38.6(B:O) IC38.9(C:I0)
N$65: IC38.3(A:O) IC38.10(C:I1)
N$66: IC42.10(C:I1) IC57.1(A:O)
N$67: IC44.13(A:I2) IC49.4(B:O)
N$69: IC42.5(B:I1) IC46.4(B:O)
N$70: IC42.2(A:I1) IC46.1(A:O)
N$72: IC44.5(B:I2) IC49.6(C:O)
N$73: IC44.11(C:I2) IC49.12(F:O)
VCC: FREIGHTERPROM1.16 FREIGHTERPROM2.16 R14.1 R15.1 R16.1 R17.1 R18.1 R19.1 R20.1 ; also sheet 5,6,8,9,10,11,14
Unconnected: IC38.11(D:O) IC38.12(D:I0) IC38.13(D:I1) IC40.3(B:I0) IC40.4(B:I1) IC40.5(B:I2) IC40.6(B:O) IC40.8(C:O) IC40.9(C:I0) IC40.10(C:I1) IC40.11(C:I2) IC42.11(D:O) IC42.12(D:I0) IC42.13(D:I1) IC46.8(C:I0) IC46.9(C:I1) IC46.10(C:O) IC46.11(D:I0) IC46.12(D:I1) IC46.13(D:O) IC47.1(A:I0) IC47.2(A:I1) IC47.4(A:I2) IC47.5(A:I3) IC47.6(A:O) IC47.8(B:O) IC47.9(B:I0) IC47.10(B:I1) IC47.12(B:I2) IC47.13(B:I3) IC49.8(D:O) IC49.9(D:I) IC49.10(E:O) IC49.11(E:I) IC50.3(B:I0) IC50.4(B:I1) IC50.5(B:I2) IC50.6(B:O) IC50.8(C:O) IC50.9(C:I0) IC50.10(C:I1) IC50.11(C:I2) IC57.4(B:O) IC57.5(B:I0) IC57.6(B:I1) IC57.8(C:I0) IC57.9(C:I1) IC57.10(C:O) IC57.11(D:I0) IC57.12(D:I1) IC57.13(D:O) U5.15(RCO)

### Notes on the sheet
- data outputs
- pullups
- Adressing inputs
- Freighter Prom #1 contains
  the top 32x8 pixels of the 
  freighter.
- Freighter Prom #2 contains
  the bottom 32x8 pixels of the 
  freighter.
- Making the full freighter graphic 
  16 x 32 pixels.
- Veritcal Line Counter,
  Top PROM enable.
- PROM bottom enable | Freighter Rom Stuff
- Check if on line 8 | Check if on line 7
- Check if on line 3 | Check if on line 6
- Check if on line 5
- Check if on line 2
- Check if on line 1 | Check if on line 4
- Data Vertical Line Selection

## Sheet 8 of 14: Submarine PROM data/addressing.
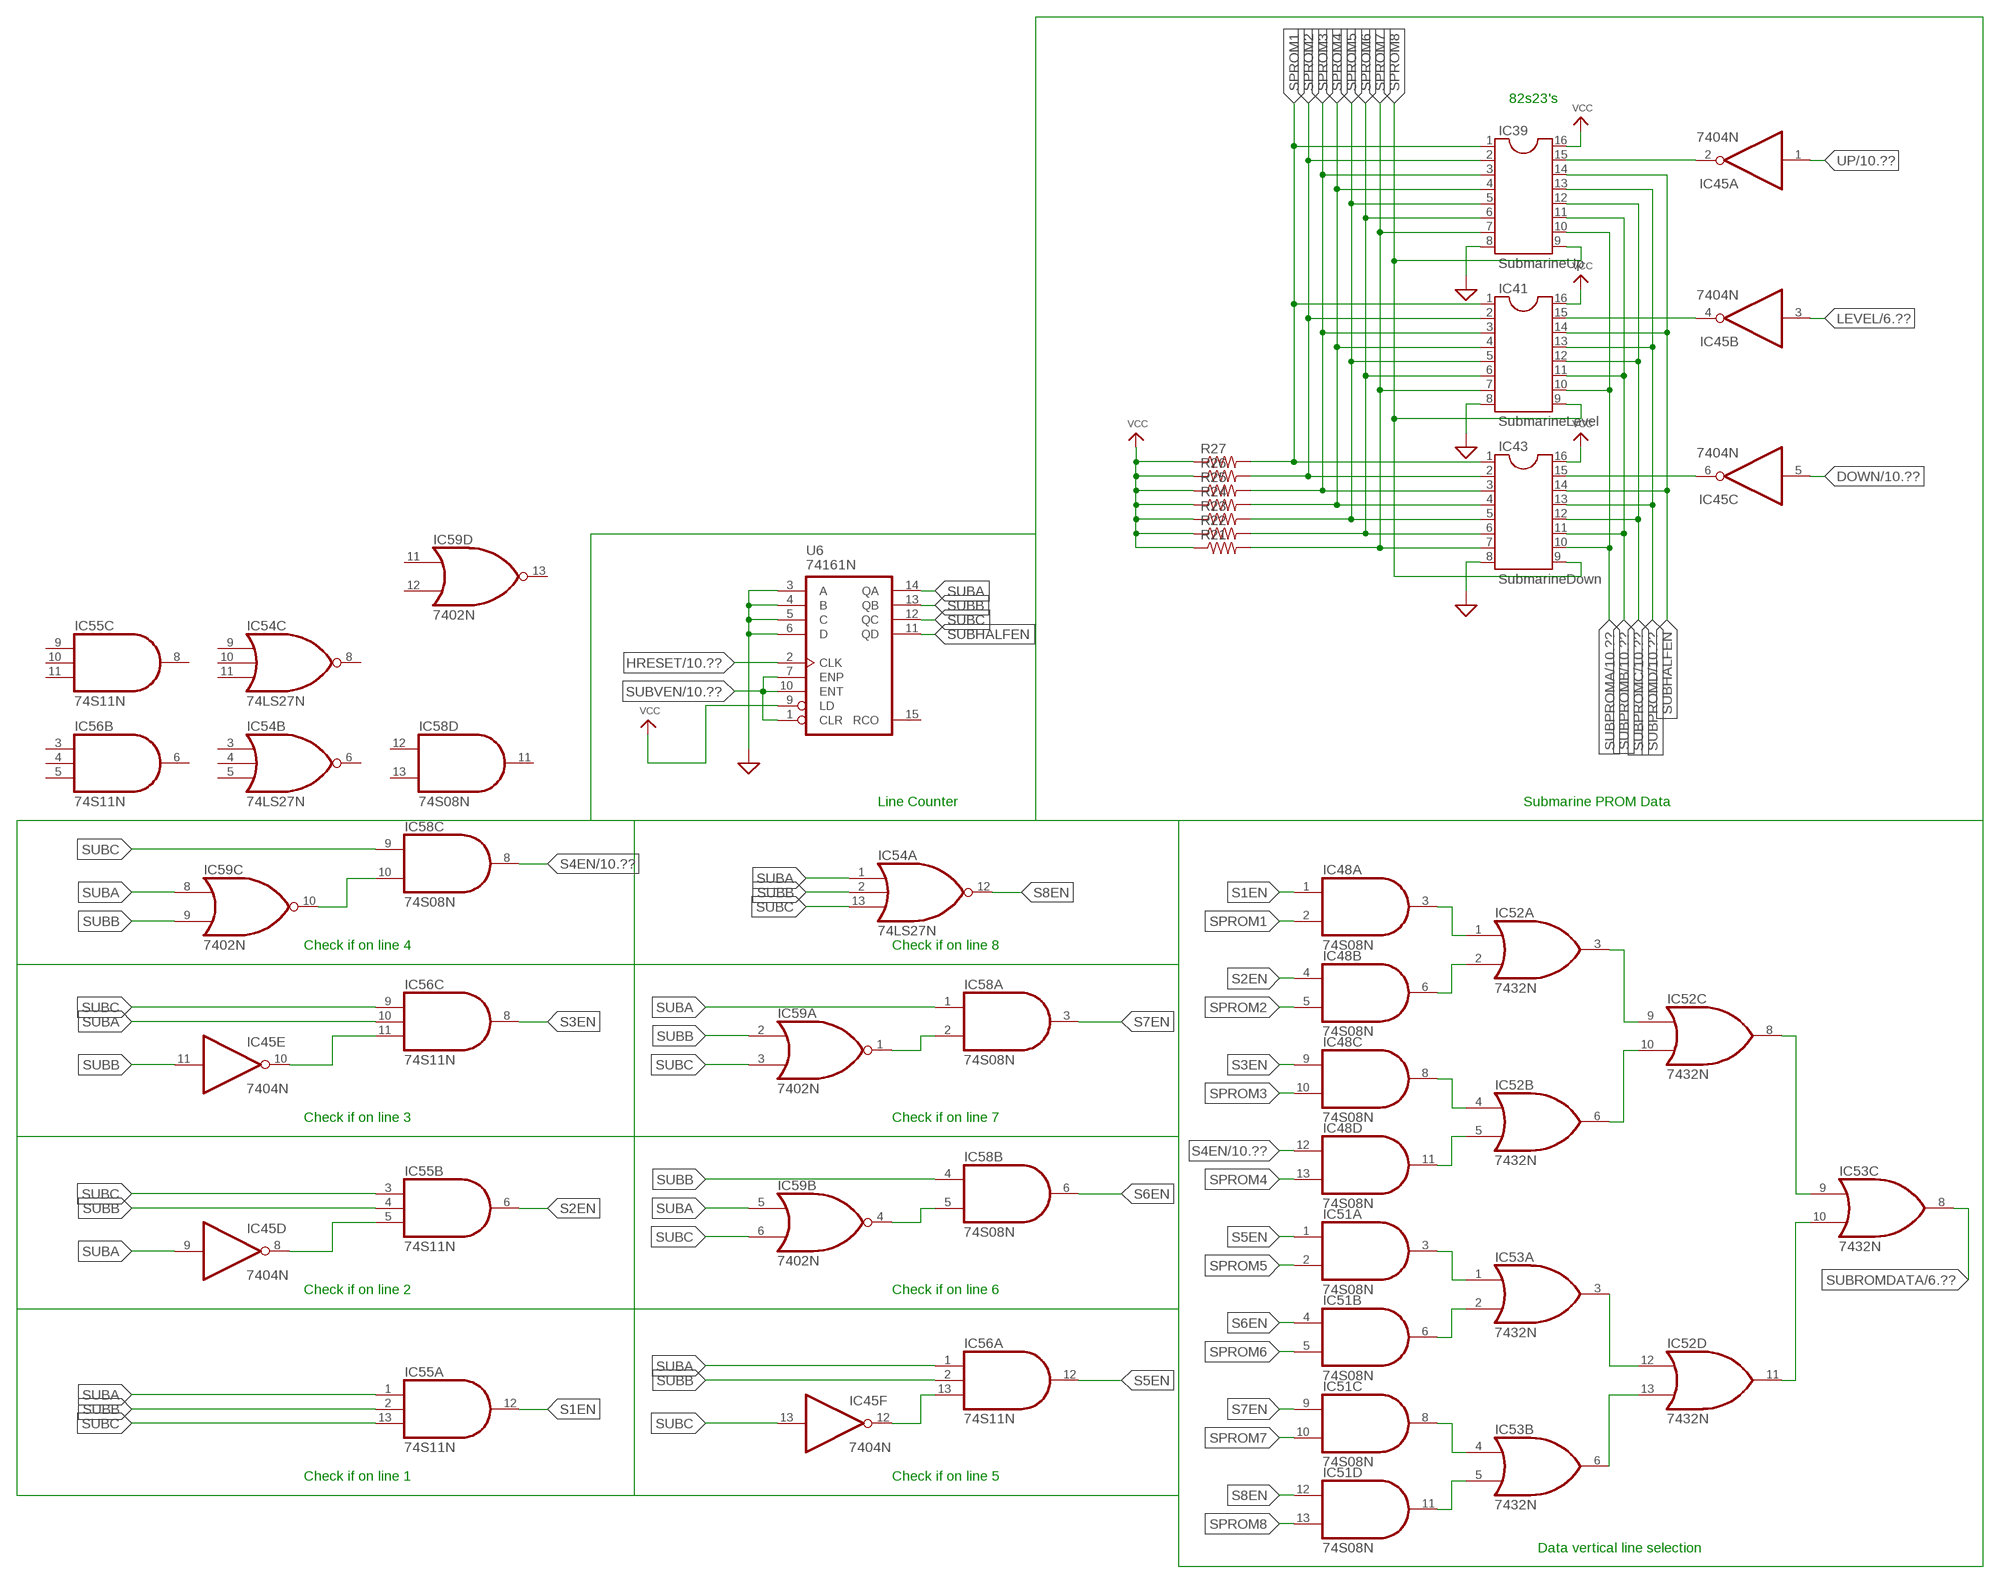
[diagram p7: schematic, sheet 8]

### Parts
IC39  SubmarineUp  DIL16S  [SOCKET-16]
IC41  SubmarineLevel  DIL16S  [SOCKET-16]
IC43  SubmarineDown  DIL16S  [SOCKET-16]
IC45  7404N  [DIL14]
IC48  74S08N  [DIL14]
IC51  74S08N  [DIL14]
IC52  7432N  [DIL14]
IC53  7432N  [DIL14]
IC54  74LS27N  [DIL14]
IC55  74S11N  [DIL14]
IC56  74S11N  [DIL14]
IC58  74S08N  [DIL14]
IC59  7402N  [DIL14]
R21  R-US_0207/10  [0207/10]
R22  R-US_0207/10  [0207/10]
R23  R-US_0207/10  [0207/10]
R24  R-US_0207/10  [0207/10]
R25  R-US_0207/10  [0207/10]
R26  R-US_0207/10  [0207/10]
R27  R-US_0207/10  [0207/10]
U6  74161N  [DIL16]

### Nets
DOWN: IC45.5(C:I) ; also sheet 6,10
GND: IC39.8 IC41.8 IC43.8 U6.3(A) U6.4(B) U6.5(C) U6.6(D) ; supply symbol labelled SUP ; also sheet 5,6,7,9,10,11,14
HRESET: U6.2(CLK) ; also sheet 1,2,7,10
LEVEL: IC45.3(B:I) ; also sheet 6
N$49: IC58.2(A:I1) IC59.1(A:O)
N$71: IC48.3(A:O) IC52.1(A:I0)
N$74: IC48.6(B:O) IC52.2(A:I1)
N$75: IC48.8(C:O) IC52.4(B:I0)
N$76: IC48.11(D:O) IC52.5(B:I1)
N$77: IC51.3(A:O) IC53.1(A:I0)
N$78: IC43.15 IC45.6(C:O)
N$79: IC41.15 IC45.4(B:O)
N$80: IC39.15 IC45.2(A:O)
N$81: IC51.6(B:O) IC53.2(A:I1)
N$82: IC51.8(C:O) IC53.4(B:I0)
N$83: IC51.11(D:O) IC53.5(B:I1)
N$84: IC52.13(D:I1) IC53.6(B:O)
N$85: IC52.12(D:I0) IC53.3(A:O)
N$86: IC52.11(D:O) IC53.10(C:I1)
N$87: IC52.6(B:O) IC52.10(C:I1)
N$88: IC52.3(A:O) IC52.9(C:I0)
N$89: IC52.8(C:O) IC53.9(C:I0)
N$90: IC58.5(B:I1) IC59.4(B:O)
N$91: IC58.10(C:I1) IC59.10(C:O)
N$92: IC45.12(F:O) IC56.13(A:I2)
N$93: IC45.10(E:O) IC56.11(C:I2)
N$94: IC45.8(D:O) IC55.5(B:I2)
S1EN: IC48.1(A:I0) IC55.12(A:O)
S2EN: IC48.4(B:I0) IC55.6(B:O)
S3EN: IC48.9(C:I0) IC56.8(C:O)
S4EN: IC48.12(D:I0) IC58.8(C:O) ; also sheet 10
S5EN: IC51.1(A:I0) IC56.12(A:O)
S6EN: IC51.4(B:I0) IC58.6(B:O)
S7EN: IC51.9(C:I0) IC58.3(A:O)
S8EN: IC51.12(D:I0) IC54.12(A:O)
SPROM1: IC39.1 IC41.1 IC43.1 IC48.2(A:I1) R27.2
SPROM2: IC39.2 IC41.2 IC43.2 IC48.5(B:I1) R26.2
SPROM3: IC39.3 IC41.3 IC43.3 IC48.10(C:I1) R25.2
SPROM4: IC39.4 IC41.4 IC43.4 IC48.13(D:I1) R24.2
SPROM5: IC39.5 IC41.5 IC43.5 IC51.2(A:I1) R23.2
SPROM6: IC39.6 IC41.6 IC43.6 IC51.5(B:I1) R22.2
SPROM7: IC39.7 IC41.7 IC43.7 IC51.10(C:I1) R21.2
SPROM8: IC39.9 IC41.9 IC43.9 IC51.13(D:I1)
SUBA: IC45.9(D:I) IC54.1(A:I0) IC55.1(A:I0) IC56.1(A:I0) IC56.10(C:I1) IC58.1(A:I0) IC59.5(B:I0) IC59.8(C:I0) U6.14(QA)
SUBB: IC45.11(E:I) IC54.2(A:I1) IC55.2(A:I1) IC55.4(B:I1) IC56.2(A:I1) IC58.4(B:I0) IC59.2(A:I0) IC59.9(C:I1) U6.13(QB)
SUBC: IC45.13(F:I) IC54.13(A:I2) IC55.3(B:I0) IC55.13(A:I2) IC56.9(C:I0) IC58.9(C:I0) IC59.3(A:I1) IC59.6(B:I1) U6.12(QC)
SUBHALFEN: IC39.14 IC41.14 IC43.14 U6.11(QD)
SUBPROMA: IC39.10 IC41.10 IC43.10 ; also sheet 6,10
SUBPROMB: IC39.11 IC41.11 IC43.11 ; also sheet 6,10
SUBPROMC: IC39.12 IC41.12 IC43.12 ; also sheet 6,10
SUBPROMD: IC39.13 IC41.13 IC43.13 ; also sheet 6,10
SUBROMDATA: IC53.8(C:O) ; also sheet 6
SUBVEN: U6.1(CLR) U6.7(ENP) U6.10(ENT) ; also sheet 6,10
UP: IC45.1(A:I) ; also sheet 6,10
VCC: IC39.16 IC41.16 IC43.16 R21.1 R22.1 R23.1 R24.1 R25.1 R26.1 R27.1 U6.9(LD) ; also sheet 5,6,7,9,10,11,14
Unconnected: IC53.11(D:O) IC53.12(D:I0) IC53.13(D:I1) IC54.3(B:I0) IC54.4(B:I1) IC54.5(B:I2) IC54.6(B:O) IC54.8(C:O) IC54.9(C:I0) IC54.10(C:I1) IC54.11(C:I2) IC55.8(C:O) IC55.9(C:I0) IC55.10(C:I1) IC55.11(C:I2) IC56.3(B:I0) IC56.4(B:I1) IC56.5(B:I2) IC56.6(B:O) IC58.11(D:O) IC58.12(D:I0) IC58.13(D:I1) IC59.11(D:I0) IC59.12(D:I1) IC59.13(D:O) U6.15(RCO)

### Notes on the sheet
- 82s23's
- Line Counter | Submarine PROM Data
- Check if on line 4 | Check if on line 8
- Check if on line 3 | Check if on line 7
- Check if on line 2 | Check if on line 6
- Check if on line 1 | Check if on line 5
- Data vertical line selection

## Sheet 9 of 14: Coin Circuitry
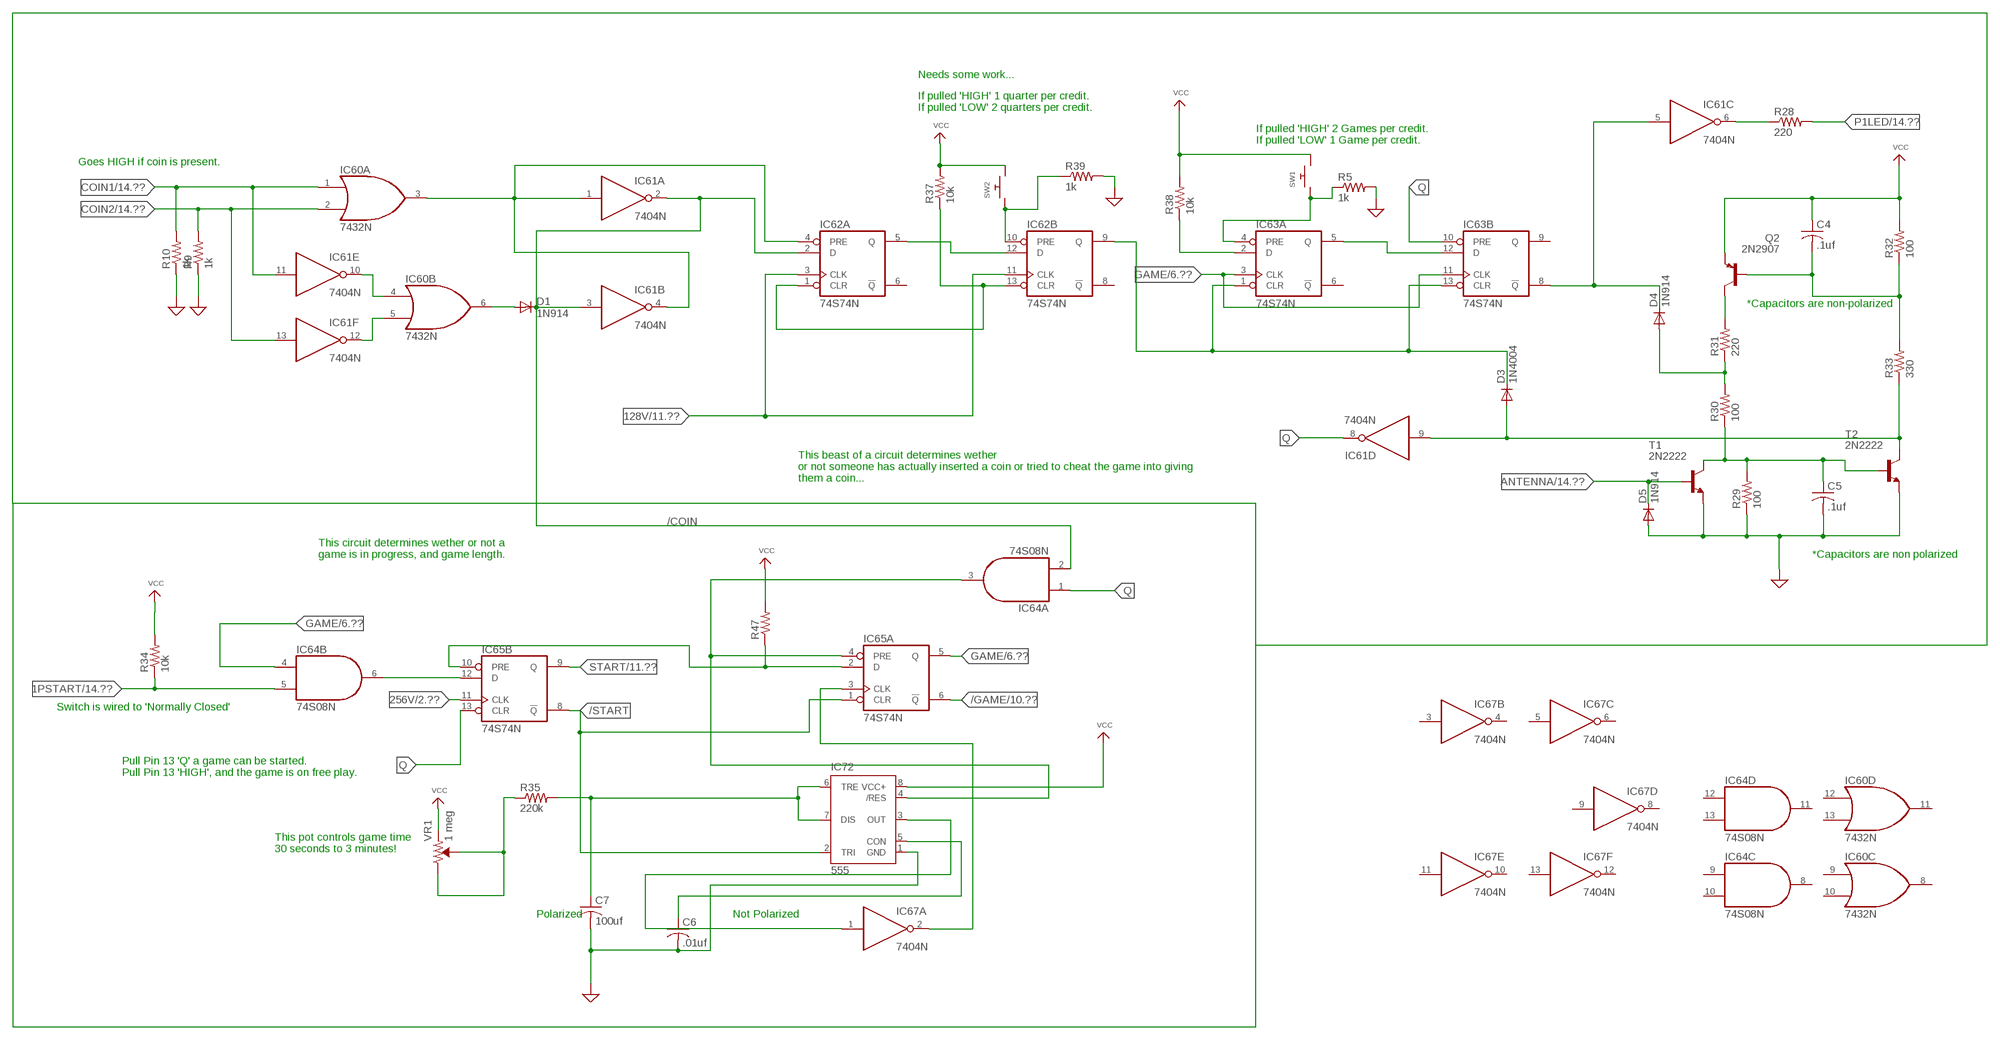
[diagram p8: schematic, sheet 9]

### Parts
C4  .1uf  C-US025-024X044  [C025-024X044]
C5  .1uf  C-US025-024X044  [C025-024X044]
C6  .01uf  C-US025-024X044  [C025-024X044]
C7  100uf  C-US025-024X044  [C025-024X044]
D1  1N914  1N4004  [DO41-10]
D3  1N4004  [DO41-10]
D4  1N914  1N4004  [DO41-10]
D5  1N914  1N4004  [DO41-10]
IC60  7432N  [DIL14]
IC61  7404N  [DIL14]
IC62  74S74N  [DIL14]
IC63  74S74N  [DIL14]
IC64  74S08N  [DIL14]
IC65  74S74N  [DIL14]
IC67  7404N  [DIL14]
IC72  555  555P  [DIP08]
Q2  2N2907  [TO92-EBC-OVAL]
R5  1k  R-US_0207/10  [0207/10]
R9  1k  R-US_0207/10  [0207/10]
R10  1k  R-US_0207/10  [0207/10]
R28  220  R-US_0207/10  [0207/10]
R29  100  R-US_0207/10  [0207/10]
R30  100  R-US_0207/10  [0207/10]
R31  220  R-US_0207/10  [0207/10]
R32  100  R-US_0207/10  [0207/10]
R33  330  R-US_0207/10  [0207/10]
R34  10k  R-US_0207/10  [0207/10]
R35  220k  R-US_0207/10  [0207/10]
R37  10k  R-US_0207/10  [0207/10]
R38  10k  R-US_0207/10  [0207/10]
R39  1k  R-US_0207/10  [0207/10]
R47  R-US_0207/10  [0207/10]
SW1  SWITCH_PUSHBUTTONEVQ-PE  [TACT_PANA-EVQ]
SW2  SWITCH_PUSHBUTTONEVQ-PE  [TACT_PANA-EVQ]
T1  2N2222  [TO92-EBC-OVAL]
T2  2N2222  [TO92-EBC-OVAL]
VR1  1 meg  TRIMPOT-PTH-10MM-KNOB-1/2W-10%  [TRIMPOT-PTH-3386U]

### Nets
1PSTART: IC64.5(B:I1) R34.1 ; also sheet 14
128V: IC62.3(A:CLK) IC62.11(B:CLK) ; also sheet 2,4,5,11
256V: IC65.11(B:CLK) ; also sheet 2
/COIN: D1.C IC61.2(A:O) IC61.3(B:I) IC62.2(A:D) IC64.2(A:I1)
/GAME: IC65.6(A:!Q) ; also sheet 6,10
/START: IC65.1(A:CLR) IC65.8(B:!Q) IC72.2(TRI)
ANTENNA: D5.C T1.B ; also sheet 14
COIN1: IC60.1(A:I0) IC61.11(E:I) R10.2 ; also sheet 14
COIN2: IC60.2(A:I1) IC61.13(F:I) R9.2 ; also sheet 14
GAME: IC63.3(A:CLK) IC63.11(B:CLK) IC64.4(B:I0) IC65.5(A:Q) ; also sheet 6
GND: C5.2 C6.2 C7.2 D5.A IC72.1(GND) R5.2 R9.1 R10.1 R29.1 R39.2 T1.E T2.E ; supply symbol labelled SUP ; also sheet 5,6,7,8,10,11,14
N$38: IC60.4(B:I0) IC61.10(E:O)
N$39: IC60.5(B:I1) IC61.12(F:O)
N$95: Q2.C R31.2
N$96: IC63.5(A:Q) IC63.12(B:D)
N$97: IC62.5(A:Q) IC62.12(B:D)
N$98: IC60.3(A:O) IC61.1(A:I) IC61.4(B:O) IC62.4(A:PRE)
N$99: D3.C IC62.9(B:Q) IC63.1(A:CLR) IC63.13(B:CLR)
N$100: IC63.4(A:PRE) R5.1 SW1.P$1
N$101: D4.C IC61.5(C:I) IC63.8(B:!Q)
N$102: IC61.6(C:O) R28.1
N$103: D4.A R30.2 R31.1
N$104: IC64.3(A:O) IC65.4(A:PRE) IC72.4(/RES)
N$105: D3.A IC61.9(D:I) R33.1 T2.C
N$106: C4.2 Q2.B R32.1 R33.2
N$107: C5.1 R29.2 R30.1 T1.C T2.B
N$108: IC64.6(B:O) IC65.12(B:D)
N$109: C6.1 IC72.5(CON)
N$111: R34.2
N$112: IC65.3(A:CLK) IC67.2(A:O)
N$114: IC67.1(A:I) IC72.3(OUT)
N$116: C7.1 IC72.6(TRE) IC72.7(DIS) R35.2
N$118: R35.1 VR1.2(WIPER) VR1.3(CW)
N$119: D1.A IC60.6(B:O)
N$120: IC62.1(A:CLR) IC62.13(B:CLR) R37.1
N$123: IC63.2(A:D) R38.1
N$124: IC62.10(B:PRE) R39.1 SW2.P$1
N$213: IC65.2(A:D) IC65.10(B:PRE) R47.1
P1LED: R28.2 ; also sheet 14
Q: IC61.8(D:O) IC63.10(B:PRE) IC64.1(A:I0) IC65.13(B:CLR)
START: IC65.9(B:Q) ; also sheet 5,6,11
VCC: C4.1 IC72.8(VCC+) Q2.E R32.2 R37.2 R38.2 R47.2 SW1.P$2 SW2.P$2 VR1.1(CCW) ; also sheet 5,6,7,8,10,11,14
Unconnected: IC60.8(C:O) IC60.9(C:I0) IC60.10(C:I1) IC60.11(D:O) IC60.12(D:I0) IC60.13(D:I1) IC62.6(A:!Q) IC62.8(B:!Q) IC63.6(A:!Q) IC63.9(B:Q) IC64.8(C:O) IC64.9(C:I0) IC64.10(C:I1) IC64.11(D:O) IC64.12(D:I0) IC64.13(D:I1) IC67.3(B:I) IC67.4(B:O) IC67.5(C:I) IC67.6(C:O) IC67.8(D:O) IC67.9(D:I) IC67.10(E:O) IC67.11(E:I) IC67.12(F:O) IC67.13(F:I)

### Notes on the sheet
- Needs some work...
- If pulled 'HIGH' 1 quarter per credit.
  If pulled 'LOW' 2 quarters per credit.
- If pulled 'HIGH' 2 Games per credit.
  If pulled 'LOW' 1 Game per credit.
- Goes HIGH if coin is present.
- *Capacitors are non-polarized
- This beast of a circuit determines wether 
  or not someone has actually inserted a coin or tried to cheat the game into giving
  them a coin...
- This circuit determines wether or not a
  game is in progress, and game length.
- *Capacitors are non polarized
- Switch is wired to 'Normally Closed'
- Pull Pin 13 'Q' a game can be started.
  Pull Pin 13 'HIGH', and the game is on free play.
- This pot controls game time
  30 seconds to 3 minutes!
- Polarized | Not Polarized

## Sheet 10 of 14: Torpedo
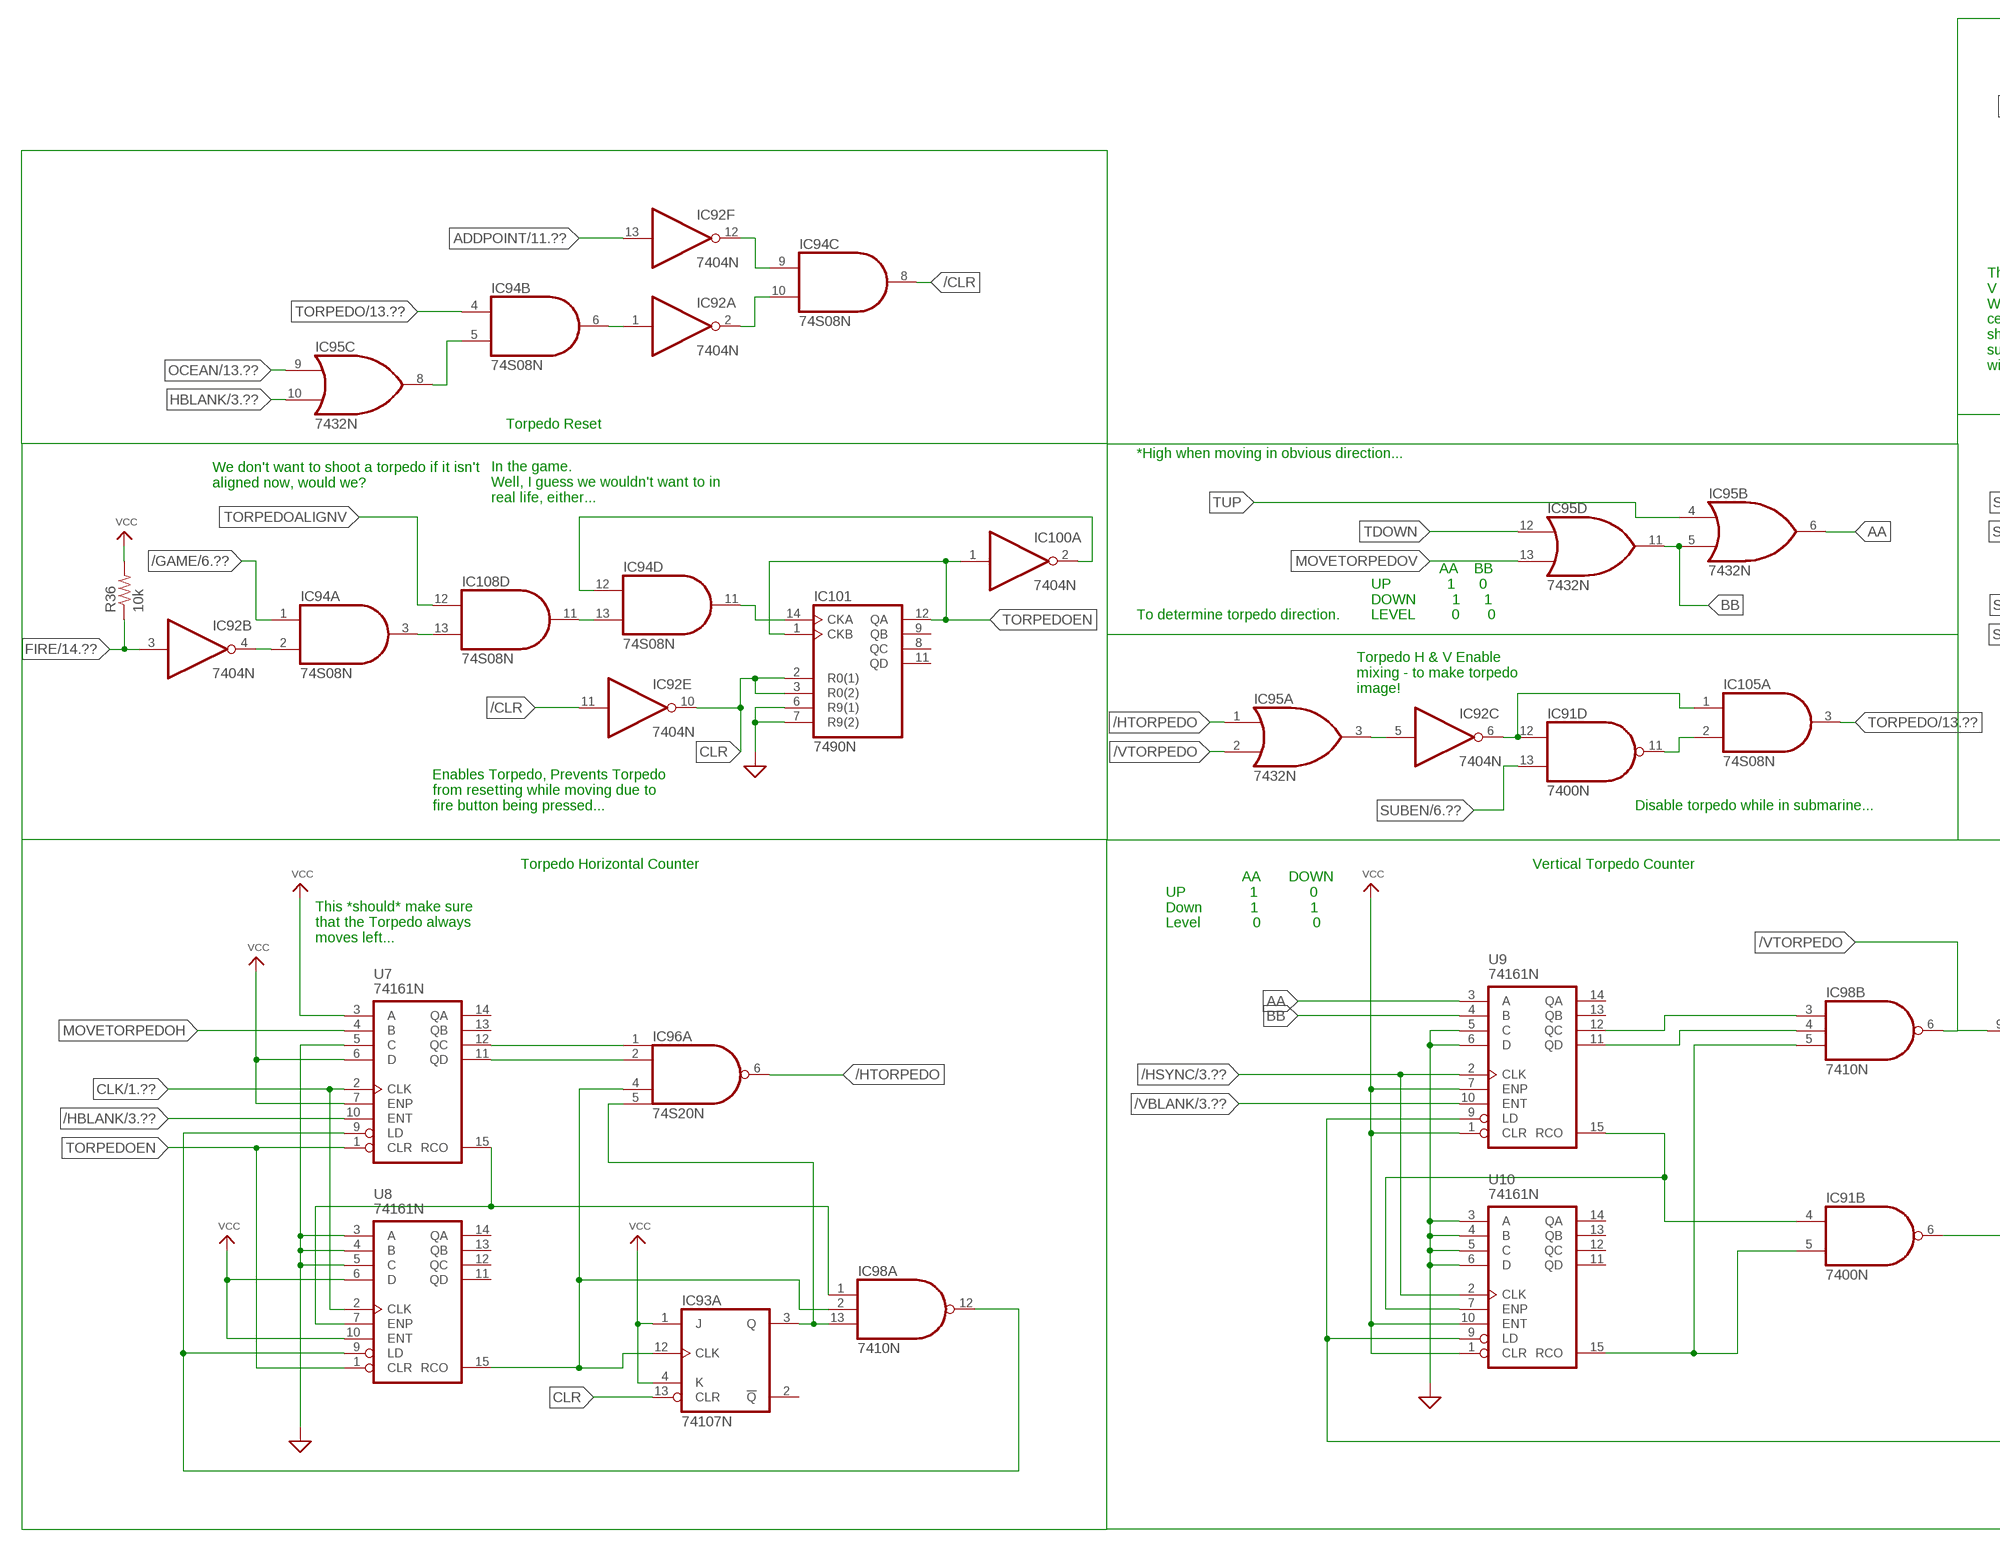
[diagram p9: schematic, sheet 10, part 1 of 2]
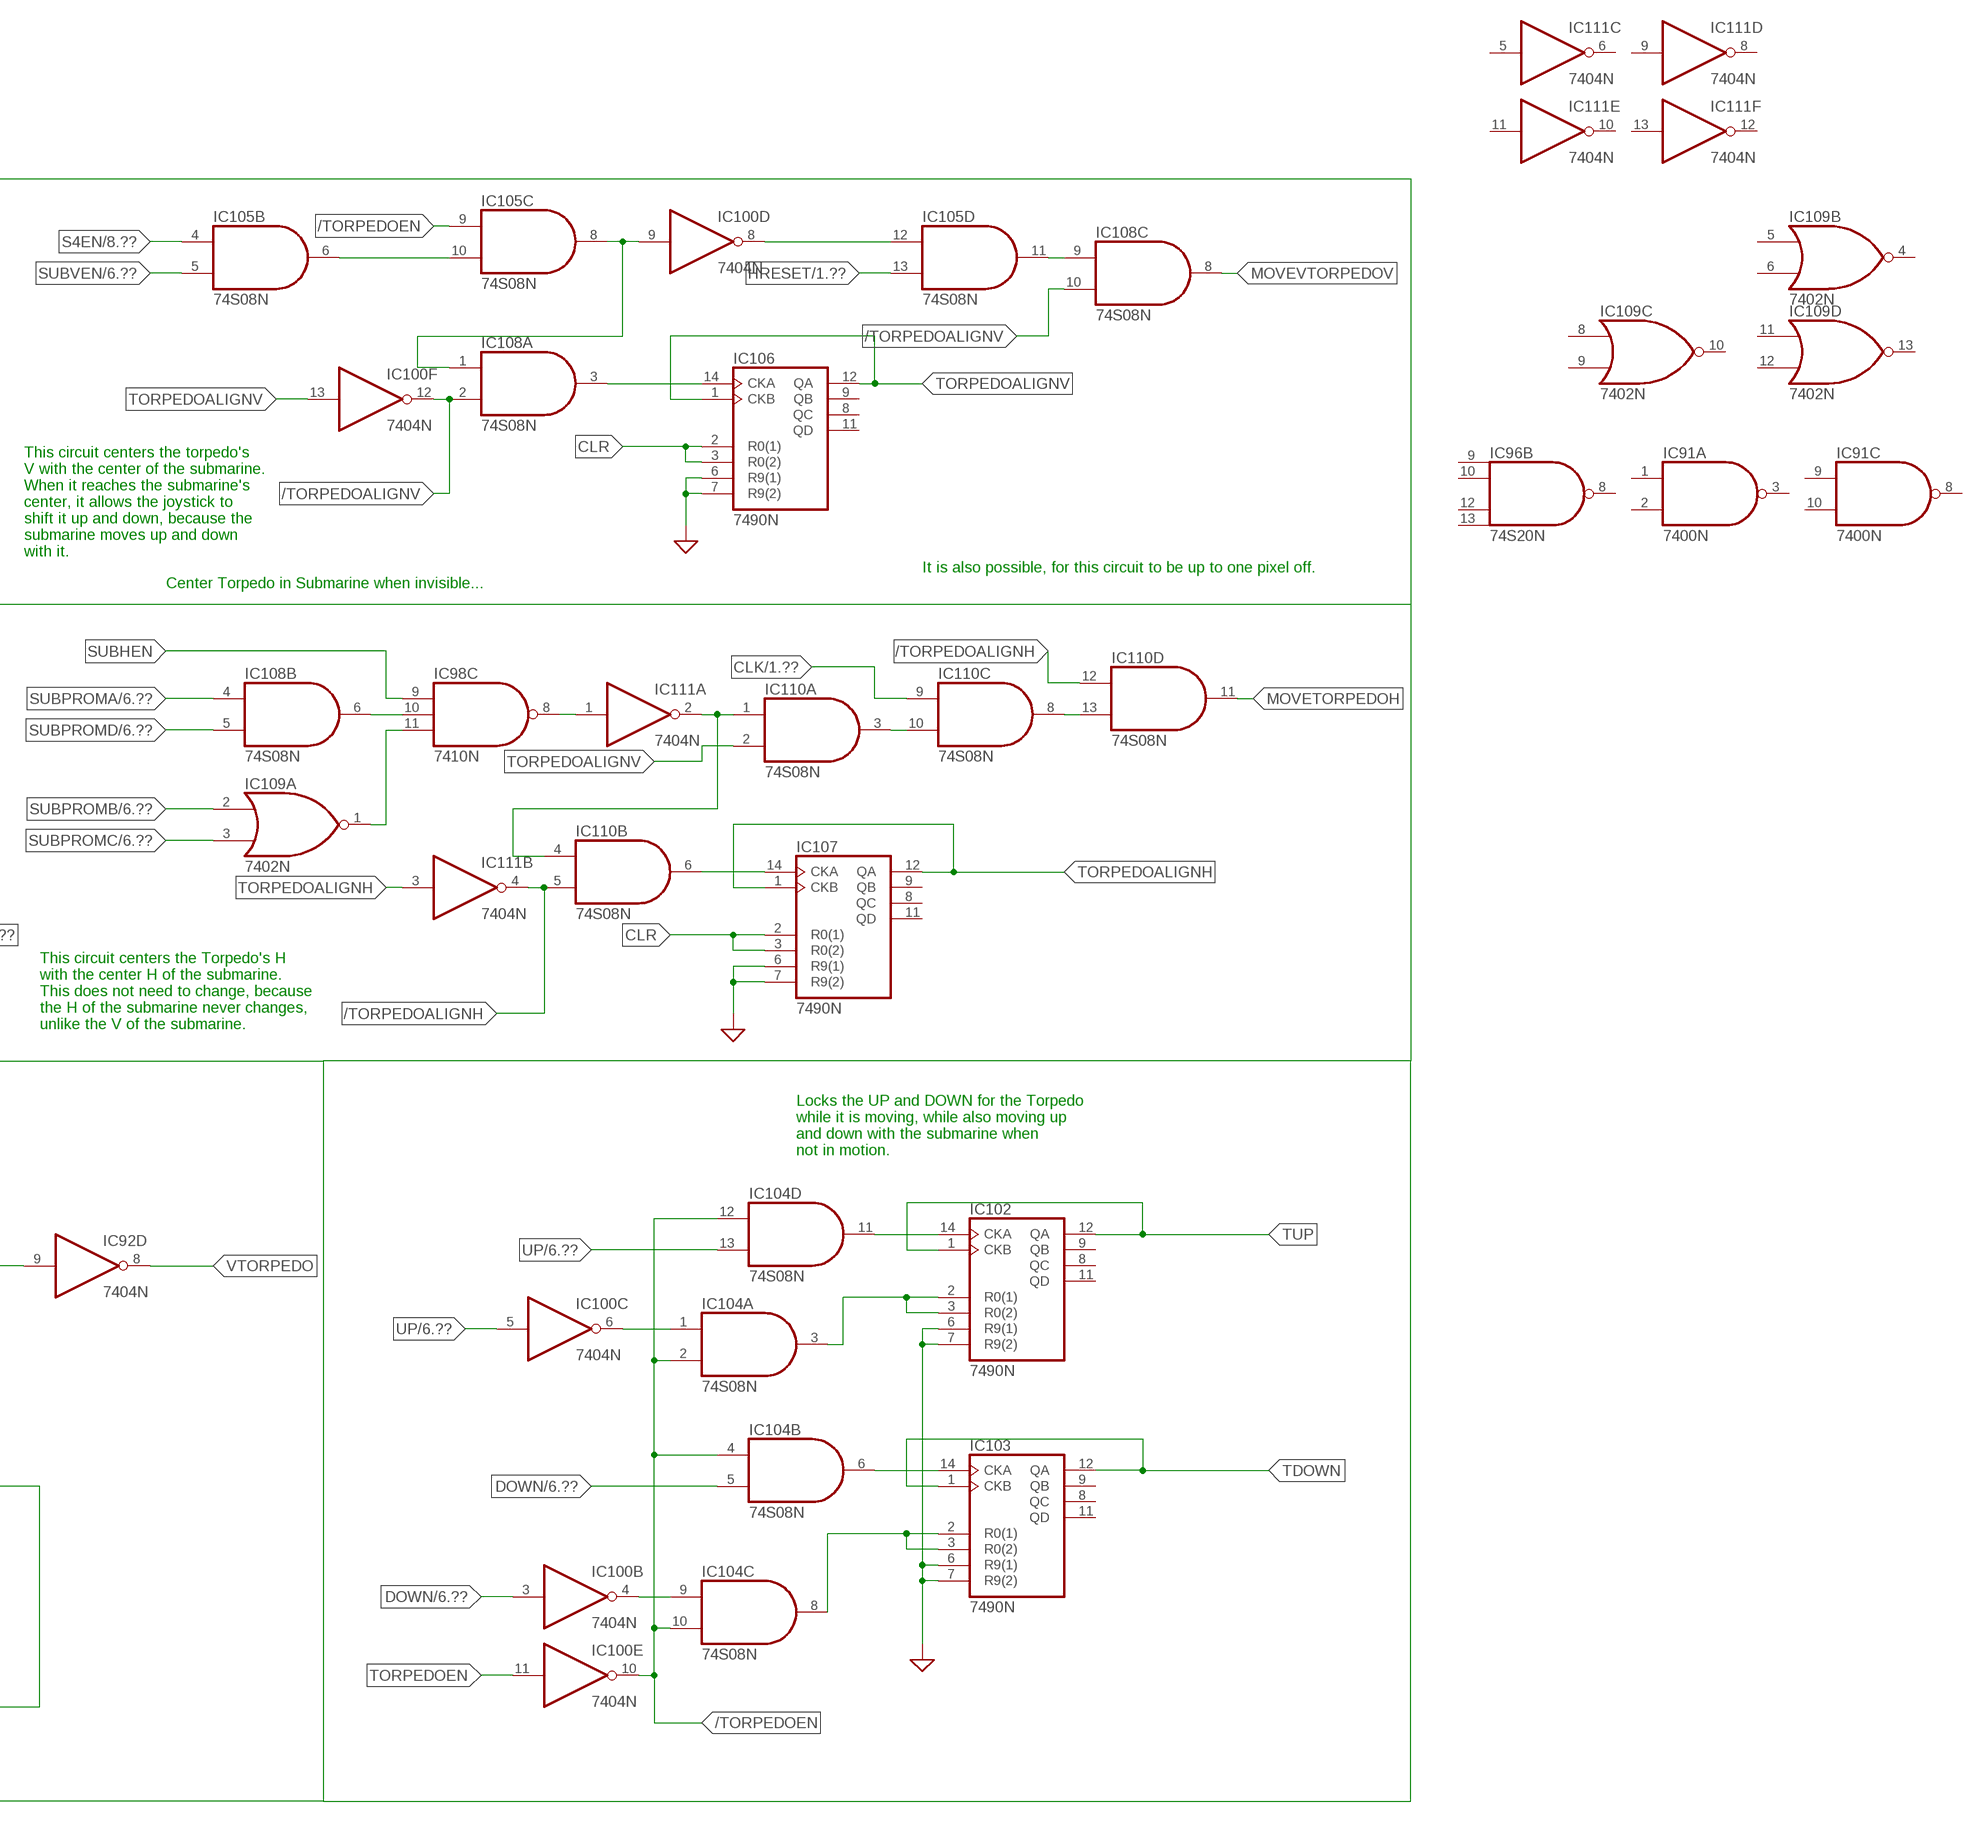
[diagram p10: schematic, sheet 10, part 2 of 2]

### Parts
IC91  7400N  [DIL14]
IC92  7404N  [DIL14]
IC93  74107N  [DIL14]
IC94  74S08N  [DIL14]
IC95  7432N  [DIL14]
IC96  74S20N  [DIL14]
IC98  7410N  [DIL14]
IC100  7404N  [DIL14]
IC101  7490N  [DIL14]
IC102  7490N  [DIL14]
IC103  7490N  [DIL14]
IC104  74S08N  [DIL14]
IC105  74S08N  [DIL14]
IC106  7490N  [DIL14]
IC107  7490N  [DIL14]
IC108  74S08N  [DIL14]
IC109  7402N  [DIL14]
IC110  74S08N  [DIL14]
IC111  7404N  [DIL14]
R36  10k  R-US_0207/10  [0207/10]
U7  74161N  [DIL16]
U8  74161N  [DIL16]
U9  74161N  [DIL16]
U10  74161N  [DIL16]

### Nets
/CLR: IC92.11(E:I) IC94.8(C:O)
/GAME: IC94.1(A:I0) ; also sheet 6,9
/HBLANK: U7.10(ENT) ; also sheet 3
/HSYNC: U9.2(CLK) U10.2(CLK) ; also sheet 3,6
/HTORPEDO: IC95.1(A:I0) IC96.6(A:O)
/TORPEDOALIGNH: IC110.5(B:I1) IC110.12(D:I0) IC111.4(B:O)
/TORPEDOALIGNV: IC100.12(F:O) IC108.2(A:I1) IC108.10(C:I1)
/TORPEDOEN: IC100.10(E:O) IC104.2(A:I1) IC104.4(B:I0) IC104.10(C:I1) IC104.12(D:I0) IC105.9(C:I0)
/VBLANK: U9.10(ENT) ; also sheet 3,6
/VTORPEDO: IC92.9(D:I) IC95.2(A:I1) IC98.6(B:O)
AA: IC95.6(B:O) U9.3(A)
ADDPOINT: IC92.13(F:I) ; also sheet 5,11
BB: IC95.5(B:I1) IC95.11(D:O) U9.4(B)
CLK: IC110.9(C:I0) U7.2(CLK) U8.2(CLK) ; also sheet 1
CLR: IC92.10(E:O) IC93.13(A:CLR) IC101.2(R0(1)) IC101.3(R0(2)) IC106.2(R0(1)) IC106.3(R0(2)) IC107.2(R0(1)) IC107.3(R0(2))
DOWN: IC100.3(B:I) IC104.5(B:I1) ; also sheet 6,8
FIRE: IC92.3(B:I) R36.1 ; also sheet 14
GND: IC101.6(R9(1)) IC101.7(R9(2)) IC102.6(R9(1)) IC102.7(R9(2)) IC103.6(R9(1)) IC103.7(R9(2)) IC106.6(R9(1)) IC106.7(R9(2)) IC107.6(R9(1)) IC107.7(R9(2)) U7.5(C) U8.3(A) U8.4(B) U8.5(C) U9.5(C) U9.6(D) U10.3(A) U10.4(B) U10.5(C) U10.6(D) ; supply symbol labelled SUP ; also sheet 5,6,7,8,9,11,14
HBLANK: IC95.10(C:I1) ; also sheet 3,5
HRESET: IC105.13(D:I1) ; also sheet 1,2,7,8
MOVETORPEDOH: IC110.11(D:O) U7.4(B)
MOVETORPEDOV: IC95.13(D:I1)
MOVEVTORPEDOV: IC108.8(C:O)
N$132: IC94.5(B:I1) IC95.8(C:O)
N$164: IC94.3(A:O) IC108.13(D:I1)
N$165: IC92.4(B:O) IC94.2(A:I1)
N$166: IC96.1(A:I0) U7.12(QC)
N$167: IC96.2(A:I1) U7.11(QD)
N$168: IC92.1(A:I) IC94.6(B:O)
N$169: IC92.12(F:O) IC94.9(C:I0)
N$171: IC92.2(A:O) IC94.10(C:I1)
N$172: IC93.3(A:Q) IC96.5(A:I3) IC98.13(A:I2)
N$175: IC93.12(A:CLK) IC96.4(A:I2) IC98.2(A:I1) U8.15(RCO)
N$176: IC98.1(A:I0) U7.15(RCO) U8.7(ENP)
N$179: IC91.4(B:I0) U9.15(RCO) U10.7(ENP)
N$180: IC98.12(A:O) U7.9(LD) U8.9(LD)
N$181: IC92.5(C:I) IC95.3(A:O)
N$182: IC94.11(D:O) IC101.14(CKA)
N$183: IC98.3(B:I0) U9.12(QC)
N$184: IC98.4(B:I1) U9.11(QD)
N$185: IC91.5(B:I1) IC98.5(B:I2) U10.15(RCO)
N$187: IC91.6(B:O) U9.9(LD) U10.9(LD)
N$188: IC94.12(D:I0) IC100.2(A:O)
N$189: IC103.2(R0(1)) IC103.3(R0(2)) IC104.8(C:O)
N$191: IC103.14(CKA) IC104.6(B:O)
N$192: IC100.6(C:O) IC104.1(A:I0)
N$193: IC91.12(D:I0) IC92.6(C:O) IC105.1(A:I0)
N$194: IC102.2(R0(1)) IC102.3(R0(2)) IC104.3(A:O)
N$195: IC102.14(CKA) IC104.11(D:O)
N$196: IC100.8(D:O) IC105.12(D:I0)
N$197: IC100.4(B:O) IC104.9(C:I0)
N$198: IC105.6(B:O) IC105.10(C:I1)
N$199: IC100.9(D:I) IC105.8(C:O) IC108.1(A:I0)
N$200: IC94.13(D:I1) IC108.11(D:O)
N$201: IC106.14(CKA) IC108.3(A:O)
N$202: IC110.1(A:I0) IC110.4(B:I0) IC111.2(A:O)
N$203: IC105.11(D:O) IC108.9(C:I0)
N$204: IC110.8(C:O) IC110.13(D:I1)
N$205: IC110.3(A:O) IC110.10(C:I1)
N$206: IC107.14(CKA) IC110.6(B:O)
N$207: IC98.10(C:I1) IC108.6(B:O)
N$208: IC98.8(C:O) IC111.1(A:I)
N$209: IC98.11(C:I2) IC109.1(A:O)
OCEAN: IC95.9(C:I0) ; also sheet 4,5,6,13
S4EN: IC105.4(B:I0) ; also sheet 8
SUBEN: IC91.13(D:I1) ; also sheet 6
SUBHEN: IC98.9(C:I0) ; also sheet 6
SUBPROMA: IC108.4(B:I0) ; also sheet 6,8
SUBPROMB: IC109.2(A:I0) ; also sheet 6,8
SUBPROMC: IC109.3(A:I1) ; also sheet 6,8
SUBPROMD: IC108.5(B:I1) ; also sheet 6,8
SUBVEN: IC105.5(B:I1) ; also sheet 6,8
TDOWN: IC95.12(D:I0) IC103.1(CKB) IC103.12(QA)
TORPEDO: IC91.11(D:O) IC94.4(B:I0) IC105.2(A:I1) IC105.3(A:O) ; also sheet 5,13
TORPEDOALIGNH: IC107.1(CKB) IC107.12(QA) IC111.3(B:I)
TORPEDOALIGNV: IC100.13(F:I) IC106.1(CKB) IC106.12(QA) IC108.12(D:I0) IC110.2(A:I1)
TORPEDOEN: IC100.1(A:I) IC100.11(E:I) IC101.1(CKB) IC101.12(QA) U7.1(CLR) U8.1(CLR)
TUP: IC95.4(B:I0) IC102.1(CKB) IC102.12(QA)
UP: IC100.5(C:I) IC104.13(D:I1) ; also sheet 6,8
VCC: IC93.1(A:J) IC93.4(A:K) R36.2 U7.3(A) U7.6(D) U7.7(ENP) U8.6(D) U8.10(ENT) U9.1(CLR) U9.7(ENP) U10.1(CLR) U10.10(ENT) ; also sheet 5,6,7,8,9,11,14
VTORPEDO: IC92.8(D:O)
Unconnected: IC91.1(A:I0) IC91.2(A:I1) IC91.3(A:O) IC91.8(C:O) IC91.9(C:I0) IC91.10(C:I1) IC93.2(A:!Q) IC93.5(B:Q) IC93.6(B:!Q) IC93.8(B:J) IC93.9(B:CLK) IC93.10(B:CLR) IC93.11(B:K) IC96.8(B:O) IC96.9(B:I0) IC96.10(B:I1) IC96.12(B:I2) IC96.13(B:I3) IC101.8(QC) IC101.9(QB) IC101.11(QD) IC102.8(QC) IC102.9(QB) IC102.11(QD) IC103.8(QC) IC103.9(QB) IC103.11(QD) IC106.8(QC) IC106.9(QB) IC106.11(QD) IC107.8(QC) IC107.9(QB) IC107.11(QD) IC109.4(B:O) IC109.5(B:I0) IC109.6(B:I1) IC109.8(C:I0) IC109.9(C:I1) IC109.10(C:O) IC109.11(D:I0) IC109.12(D:I1) IC109.13(D:O) IC111.5(C:I) IC111.6(C:O) IC111.8(D:O) IC111.9(D:I) IC111.10(E:O) IC111.11(E:I) IC111.12(F:O) IC111.13(F:I) U7.13(QB) U7.14(QA) U8.11(QD) U8.12(QC) U8.13(QB) U8.14(QA) U9.13(QB) U9.14(QA) U10.11(QD) U10.12(QC) U10.13(QB) U10.14(QA)

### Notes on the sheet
- This circuit centers the torpedo's 
  V with the center of the submarine.
  When it reaches the submarine's
  center, it allows the joystick to 
  shift it up and down, because the 
  submarine moves up and down
  with it.
- It is also possible, for this circuit to be up to one pixel off.
- Center Torpedo in Submarine when invisible...
- Torpedo Reset
- *High when moving in obvious direction...
- We don't want to shoot a torpedo if it isn't
  aligned now, would we?
- In the game.
  Well, I guess we wouldn't want to in
  real life, either...
- To determine torpedo direction.
- AA    BB
  UP              1      0
  DOWN         1      1 
  LEVEL         0       0
- Torpedo H & V Enable
  mixing - to make torpedo
  image!
- Enables Torpedo, Prevents Torpedo
  from resetting while moving due to
  fire button being pressed...
- Disable torpedo while in submarine...
- This circuit centers the Torpedo's H
  with the center H of the submarine.
  This does not need to change, because
  the H of the submarine never changes,
  unlike the V of the submarine.
- Torpedo Horizontal Counter | Vertical Torpedo Counter
- AA       DOWN
  UP                1             0
  Down            1             1
  Level             0             0
- Locks the UP and DOWN for the Torpedo
  while it is moving, while also moving up 
  and down with the submarine when
  not in motion.
- This *should* make sure
  that the Torpedo always
  moves left...

## Sheet 11 of 14: Score
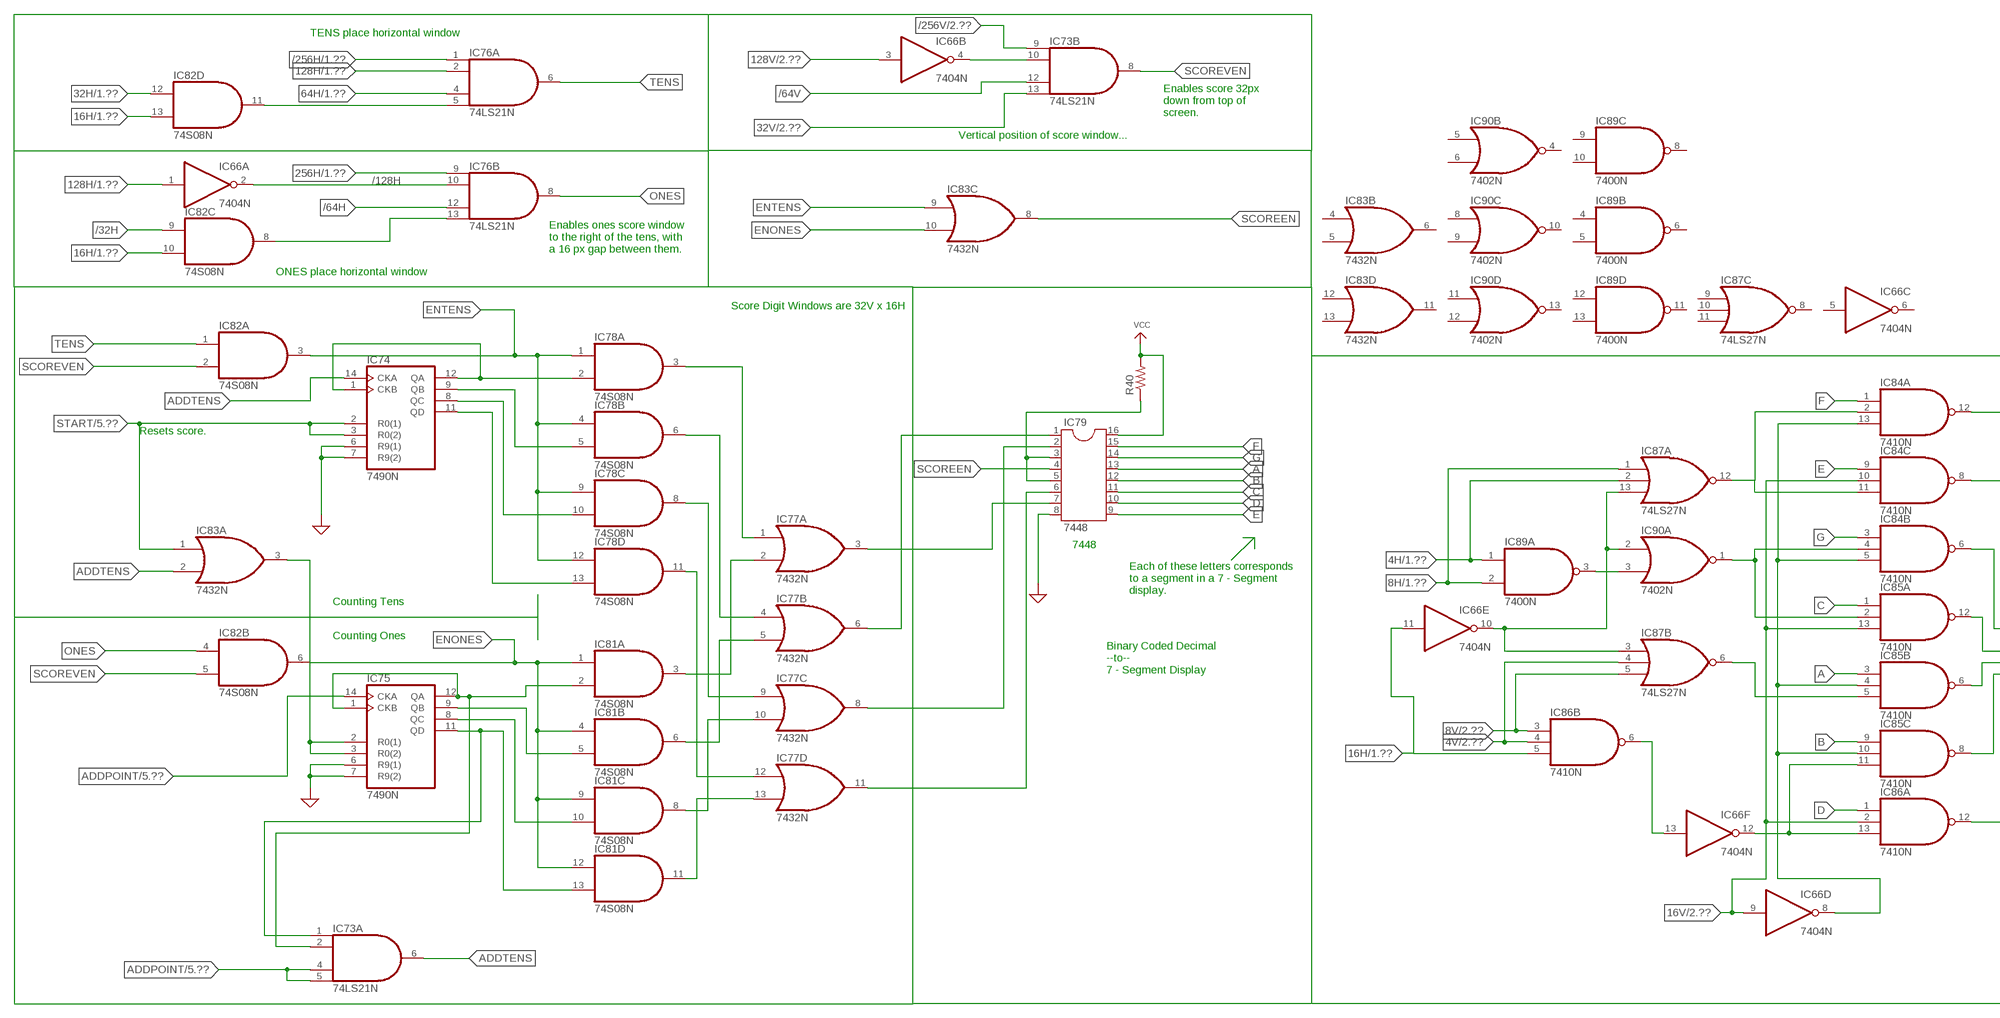
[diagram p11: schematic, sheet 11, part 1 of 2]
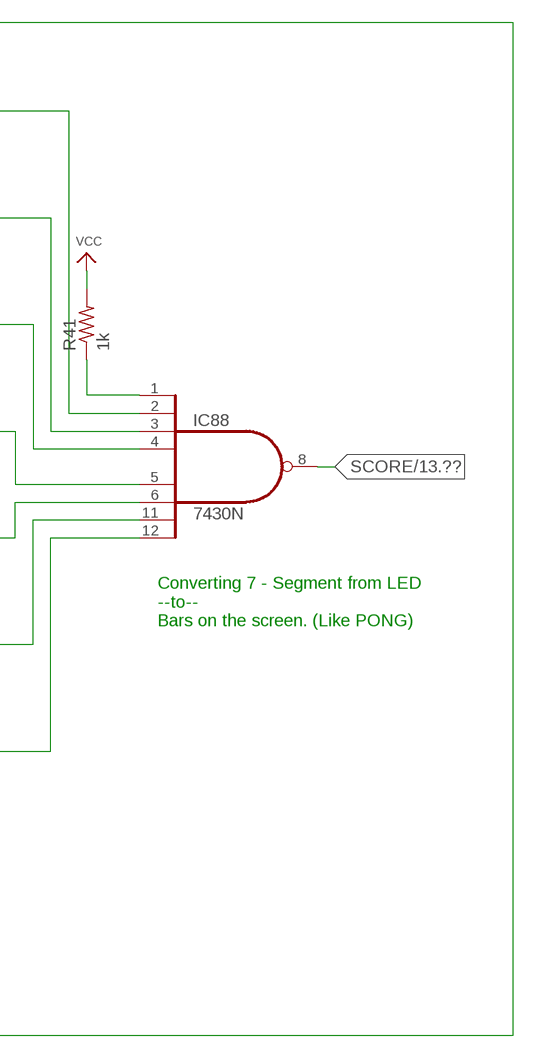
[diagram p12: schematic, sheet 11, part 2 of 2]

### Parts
IC66  7404N  [DIL14]
IC73  74LS21N  [DIL14]
IC74  7490N  [DIL14]
IC75  7490N  [DIL14]
IC76  74LS21N  [DIL14]
IC77  7432N  [DIL14]
IC78  74S08N  [DIL14]
IC79  7448  DIL16S  [SOCKET-16]
IC81  74S08N  [DIL14]
IC82  74S08N  [DIL14]
IC83  7432N  [DIL14]
IC84  7410N  [DIL14]
IC85  7410N  [DIL14]
IC86  7410N  [DIL14]
IC87  74LS27N  [DIL14]
IC88  7430N  [DIL14]
IC89  7400N  [DIL14]
IC90  7402N  [DIL14]
R40  R-US_0207/10  [0207/10]
R41  1k  R-US_0207/10  [0207/10]

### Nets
4H: IC87.2(A:I1) IC89.1(A:I0) ; also sheet 1
4V: IC86.4(B:I1) IC87.4(B:I1) ; also sheet 2,3,4
8H: IC87.1(A:I0) IC89.2(A:I1) ; also sheet 1
8V: IC86.3(B:I0) IC87.5(B:I2) ; also sheet 2,3,4
16H: IC66.11(E:I) IC82.10(C:I1) IC82.13(D:I1) IC86.5(B:I2) ; also sheet 1,3,6
16V: IC66.9(D:I) IC84.10(C:I1) IC85.13(A:I2) IC86.2(A:I1) ; also sheet 2,3,4,5
32H: IC82.12(D:I0) ; also sheet 1,3,6
32V: IC73.13(B:I3) ; also sheet 2,4,5
64H: IC76.4(A:I2) ; also sheet 1,3,6
128H: IC66.1(A:I) IC76.2(A:I1) ; also sheet 1,6
128V: IC66.3(B:I) ; also sheet 2,4,5,9
256H: IC76.9(B:I0) ; also sheet 1,6
/32H: IC82.9(C:I0) ; also sheet 6
/64H: IC76.12(B:I2) ; also sheet 6
/64V: IC73.12(B:I2) ; also sheet 4
/128H: IC66.2(A:O) IC76.10(B:I1)
/256H: IC76.1(A:I0) ; also sheet 1
/256V: IC73.9(B:I0) ; also sheet 2
A: IC79.13 IC85.3(B:I0)
ADDPOINT: IC73.4(A:I2) IC73.5(A:I3) IC75.14(CKA) ; also sheet 5,10
ADDTENS: IC73.6(A:O) IC74.14(CKA) IC83.2(A:I1)
B: IC79.12 IC85.9(C:I0)
C: IC79.11 IC85.1(A:I0)
D: IC79.10 IC86.1(A:I0)
E: IC79.9 IC84.9(C:I0)
ENONES: IC81.1(A:I0) IC81.4(B:I0) IC81.9(C:I0) IC81.12(D:I0) IC82.6(B:O) IC83.10(C:I1)
ENTENS: IC78.1(A:I0) IC78.4(B:I0) IC78.9(C:I0) IC78.12(D:I0) IC82.3(A:O) IC83.9(C:I0)
F: IC79.15 IC84.1(A:I0)
G: IC79.14 IC84.3(B:I0)
GND: IC74.6(R9(1)) IC74.7(R9(2)) IC75.6(R9(1)) IC75.7(R9(2)) IC79.8 ; supply symbol labelled SUP ; also sheet 5,6,7,8,9,10,14
N$14: IC75.9(QB) IC81.5(B:I1)
N$33: IC77.3(A:O) IC79.7
N$125: IC74.1(CKB) IC74.12(QA) IC78.2(A:I1)
N$126: IC76.13(B:I3) IC82.8(C:O)
N$127: IC66.13(F:I) IC86.6(B:O)
N$128: IC74.9(QB) IC78.5(B:I1)
N$129: IC74.8(QC) IC78.10(C:I1)
N$130: IC74.11(QD) IC78.13(D:I1)
N$131: IC73.2(A:I1) IC75.1(CKB) IC75.12(QA) IC81.2(A:I1)
N$133: IC75.8(QC) IC81.10(C:I1)
N$134: IC73.1(A:I0) IC75.11(QD) IC81.13(D:I1)
N$135: IC77.1(A:I0) IC78.3(A:O)
N$136: IC77.4(B:I0) IC78.6(B:O)
N$137: IC77.9(C:I0) IC78.8(C:O)
N$138: IC77.2(A:I1) IC81.3(A:O)
N$139: IC77.5(B:I1) IC81.6(B:O)
N$140: IC77.10(C:I1) IC81.8(C:O)
N$141: IC77.12(D:I0) IC78.11(D:O)
N$142: IC77.13(D:I1) IC81.11(D:O)
N$143: IC75.2(R0(1)) IC75.3(R0(2)) IC83.3(A:O)
N$144: IC77.6(B:O) IC79.1
N$145: IC77.8(C:O) IC79.2
N$146: IC79.6
N$147: IC84.12(A:O) IC88.2(I1)
N$148: IC84.8(C:O) IC88.3(I2)
N$149: IC84.6(B:O) IC88.4(I3)
N$150: IC85.12(A:O) IC88.5(I4)
N$151: IC85.6(B:O) IC88.6(I5)
N$152: IC85.8(C:O) IC88.11(I6)
N$153: IC86.12(A:O) IC88.12(I7)
N$154: IC79.3 IC79.5 R40.1
N$156: IC88.1(I0) R41.1
N$161: IC84.2(A:I1) IC84.11(C:I2) IC87.12(A:O)
N$162: IC66.10(E:O) IC87.3(B:I0) IC87.13(A:I2) IC90.2(A:I0)
N$163: IC89.3(A:O) IC90.3(A:I1)
N$170: IC84.4(B:I1) IC85.2(A:I1) IC90.1(A:O)
N$173: IC66.8(D:O) IC84.5(B:I2) IC84.13(A:I2) IC85.4(B:I1) IC85.10(C:I1)
N$174: IC85.5(B:I2) IC87.6(B:O)
N$177: IC66.12(F:O) IC85.11(C:I2) IC86.13(A:I2)
N$211: IC76.5(A:I3) IC82.11(D:O)
N$212: IC66.4(B:O) IC73.10(B:I1)
ONES: IC76.8(B:O) IC82.4(B:I0)
SCORE: IC88.8(O) ; also sheet 13
SCOREEN: IC79.4 IC83.8(C:O)
SCOREVEN: IC73.8(B:O) IC82.2(A:I1) IC82.5(B:I1)
START: IC74.2(R0(1)) IC74.3(R0(2)) IC83.1(A:I0) ; also sheet 5,6,9
TENS: IC76.6(A:O) IC82.1(A:I0)
VCC: IC79.16 R40.2 R41.2 ; also sheet 5,6,7,8,9,10,14
Unconnected: IC66.5(C:I) IC66.6(C:O) IC77.11(D:O) IC83.4(B:I0) IC83.5(B:I1) IC83.6(B:O) IC83.11(D:O) IC83.12(D:I0) IC83.13(D:I1) IC86.8(C:O) IC86.9(C:I0) IC86.10(C:I1) IC86.11(C:I2) IC87.8(C:O) IC87.9(C:I0) IC87.10(C:I1) IC87.11(C:I2) IC89.4(B:I0) IC89.5(B:I1) IC89.6(B:O) IC89.8(C:O) IC89.9(C:I0) IC89.10(C:I1) IC89.11(D:O) IC89.12(D:I0) IC89.13(D:I1) IC90.4(B:O) IC90.5(B:I0) IC90.6(B:I1) IC90.8(C:I0) IC90.9(C:I1) IC90.10(C:O) IC90.11(D:I0) IC90.12(D:I1) IC90.13(D:O)

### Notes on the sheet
- TENS place horizontal window
- Enables score 32px
  down from top of
  screen.
- Vertical position of score window...
- Enables ones score window
  to the right of the tens, with
  a 16 px gap between them.
- ONES place horizontal window
- Score Digit Windows are 32V x 16H
- Resets score.
- 7448
- Each of these letters corresponds
  to a segment in a 7 - Segment 
  display.
- Counting Tens
- Counting Ones
- Binary Coded Decimal 
  --to--
  7 - Segment Display
- Converting 7 - Segment from LED
  --to--
  Bars on the screen. (Like PONG)

## Sheet 12 of 14: Sound

## Sheet 13 of 14: RGB Out
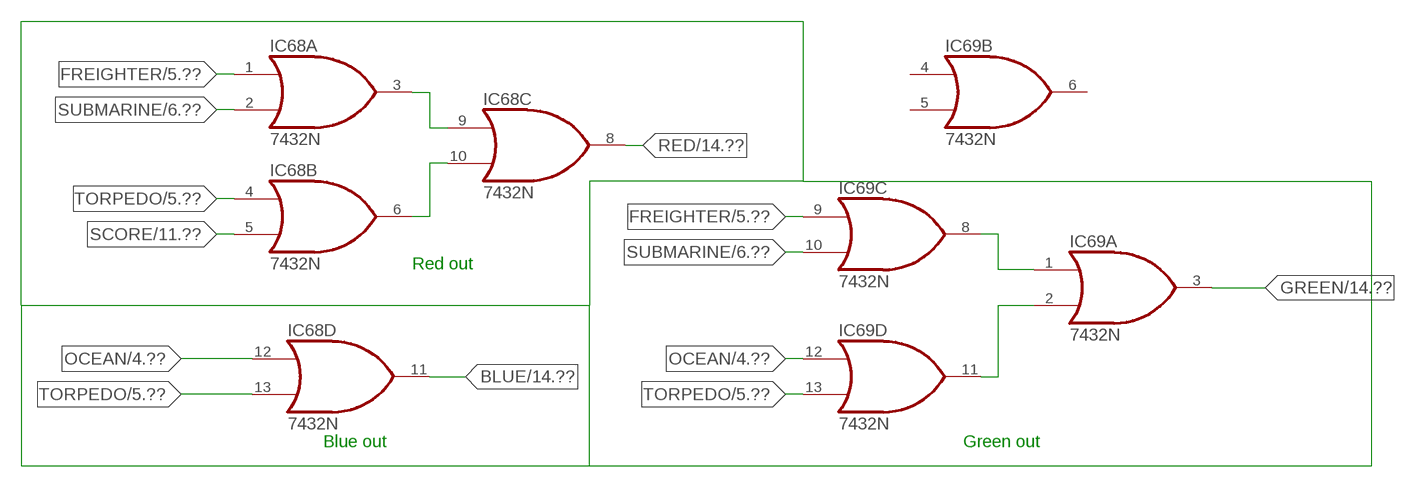
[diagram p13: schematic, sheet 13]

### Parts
IC68  7432N  [DIL14]
IC69  7432N  [DIL14]

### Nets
BLUE: IC68.11(D:O) ; also sheet 14
FREIGHTER: IC68.1(A:I0) IC69.9(C:I0) ; also sheet 5
GREEN: IC69.3(A:O) ; also sheet 14
N$115: IC68.3(A:O) IC68.9(C:I0)
N$117: IC68.6(B:O) IC68.10(C:I1)
N$121: IC69.2(A:I1) IC69.11(D:O)
N$122: IC69.1(A:I0) IC69.8(C:O)
OCEAN: IC68.12(D:I0) IC69.12(D:I0) ; also sheet 4,5,6,10
RED: IC68.8(C:O) ; also sheet 14
SCORE: IC68.5(B:I1) ; also sheet 11
SUBMARINE: IC68.2(A:I1) IC69.10(C:I1) ; also sheet 6
TORPEDO: IC68.4(B:I0) IC68.13(D:I1) IC69.13(D:I1) ; also sheet 5,10
Unconnected: IC69.4(B:I0) IC69.5(B:I1) IC69.6(B:O)

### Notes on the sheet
- Red out
- Blue out | Green out

## Sheet 14 of 14: Card Edge Connector
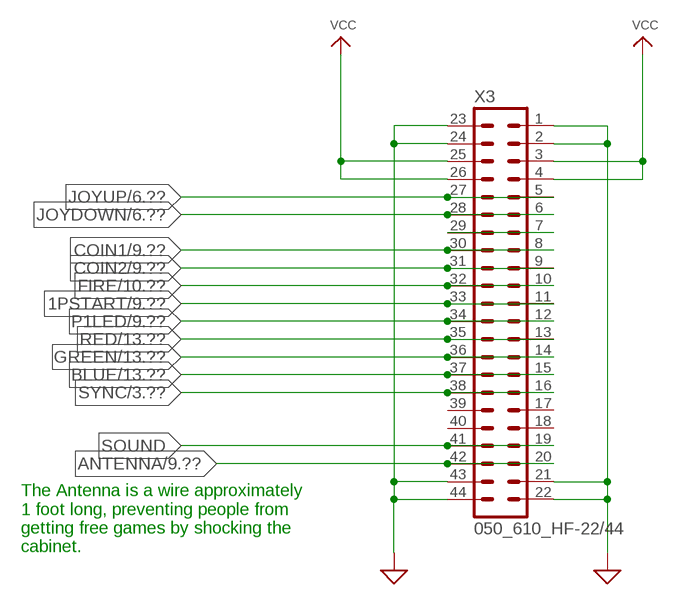
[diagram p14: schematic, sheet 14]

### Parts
X3  050_610_HF-22/44  [050_610_HF-22/44]

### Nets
1PSTART: X3.11 X3.33 ; also sheet 9
ANTENNA: X3.20 X3.42 ; also sheet 9
BLUE: X3.15 X3.37 ; also sheet 13
COIN1: X3.8 X3.30 ; also sheet 9
COIN2: X3.9 X3.31 ; also sheet 9
FIRE: X3.10 X3.32 ; also sheet 10
GND: X3.1 X3.2 X3.21 X3.22 X3.23 X3.24 X3.43 X3.44 ; supply symbol labelled SUP ; also sheet 5,6,7,8,9,10,11
GREEN: X3.14 X3.36 ; also sheet 13
JOYDOWN: X3.6 X3.28 ; also sheet 6
JOYUP: X3.5 X3.27 ; also sheet 6
N$110: X3.7 X3.29
P1LED: X3.12 X3.34 ; also sheet 9
RED: X3.13 X3.35 ; also sheet 13
SOUND: X3.19 X3.41
SYNC: X3.16 X3.38 ; also sheet 3
VCC: X3.3 X3.4 X3.25 X3.26 ; also sheet 5,6,7,8,9,10,11
Unconnected: X3.17 X3.18 X3.39 X3.40

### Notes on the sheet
- The Antenna is a wire approximately
  1 foot long, preventing people from
  getting free games by shocking the
  cabinet.

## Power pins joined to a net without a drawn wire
GND: IC1.7(P:GND) IC2.7(P:GND) IC3.7(P:GND) IC4.10(GND) IC5.10(GND) IC6.7(GND) IC7.7(GND) IC8.7(P:GND) IC9.10(GND) IC10.10(GND) IC11.7(P:GND) IC12.7(P:GND) IC13.7(P:GND) IC14.7(P:GND) IC15.7(P:GND) IC16.7(P:GND) IC17.7(P:GND) IC18.7(P:GND) IC19.7(P:GND) IC20.7(P:GND) IC21.7(P:GND) IC22.7(P:GND) IC23.7(P:GND) IC24.7(GND) IC25.7(P:GND) IC26.7(P:GND) IC27.7(P:GND) IC28.7(P:GND) IC29.7(GND) IC30.7(P:GND) IC31.7(P:GND) IC32.7(P:GND) IC33.7(P:GND) IC34.7(P:GND) IC35.7(P:GND) IC36.7(P:GND) IC37.7(P:GND) IC38.7(P:GND) IC40.7(P:GND) IC42.7(P:GND) IC44.7(P:GND) IC45.7(P:GND) IC46.7(P:GND) IC47.7(P:GND) IC48.7(P:GND) IC49.7(P:GND) IC50.7(P:GND) IC51.7(P:GND) IC52.7(P:GND) IC53.7(P:GND) IC54.7(P:GND) IC55.7(P:GND) IC56.7(P:GND) IC57.7(P:GND) IC58.7(P:GND) IC59.7(P:GND) IC60.7(P:GND) IC61.7(P:GND) IC62.7(P:GND) IC63.7(P:GND) IC64.7(P:GND) IC65.7(P:GND) IC66.7(P:GND) IC67.7(P:GND) IC68.7(P:GND) IC69.7(P:GND) IC70.7(P:GND) IC71.7(P:GND) IC73.7(P:GND) IC74.10(GND) IC75.10(GND) IC76.7(P:GND) IC77.7(P:GND) IC78.7(P:GND) IC81.7(P:GND) IC82.7(P:GND) IC83.7(P:GND) IC84.7(P:GND) IC85.7(P:GND) IC86.7(P:GND) IC87.7(P:GND) IC88.7(GND) IC89.7(P:GND) IC90.7(P:GND) IC91.7(P:GND) IC92.7(P:GND) IC93.7(P:GND) IC94.7(P:GND) IC95.7(P:GND) IC96.7(P:GND) IC97.7(P:GND) IC98.7(P:GND) IC99.7(P:GND) IC100.7(P:GND) IC101.10(GND) IC102.10(GND) IC103.10(GND) IC104.7(P:GND) IC105.7(P:GND) IC106.10(GND) IC107.10(GND) IC108.7(P:GND) IC109.7(P:GND) IC110.7(P:GND) IC111.7(P:GND) U1.8(GND) U2.8(GND) U3.8(GND) U4.8(GND) U5.8(GND) U6.8(GND) U7.8(GND) U8.8(GND) U9.8(GND) U10.8(GND)
VCC: IC1.14(P:VCC) IC2.14(P:VCC) IC3.14(P:VCC) IC4.5(VCC) IC5.5(VCC) IC6.14(VCC) IC7.14(VCC) IC8.14(P:VCC) IC9.5(VCC) IC10.5(VCC) IC11.14(P:VCC) IC12.14(P:VCC) IC13.14(P:VCC) IC14.14(P:VCC) IC15.14(P:VCC) IC16.14(P:VCC) IC17.14(P:VCC) IC18.14(P:VCC) IC19.14(P:VCC) IC20.14(P:VCC) IC21.14(P:VCC) IC22.14(P:VCC) IC23.14(P:VCC) IC24.14(VCC) IC25.14(P:VCC) IC26.14(P:VCC) IC27.14(P:VCC) IC28.14(P:VCC) IC29.14(VCC) IC30.14(P:VCC) IC31.14(P:VCC) IC32.14(P:VCC) IC33.14(P:VCC) IC34.14(P:VCC) IC35.14(P:VCC) IC36.14(P:VCC) IC37.14(P:VCC) IC38.14(P:VCC) IC40.14(P:VCC) IC42.14(P:VCC) IC44.14(P:VCC) IC45.14(P:VCC) IC46.14(P:VCC) IC47.14(P:VCC) IC48.14(P:VCC) IC49.14(P:VCC) IC50.14(P:VCC) IC51.14(P:VCC) IC52.14(P:VCC) IC53.14(P:VCC) IC54.14(P:VCC) IC55.14(P:VCC) IC56.14(P:VCC) IC57.14(P:VCC) IC58.14(P:VCC) IC59.14(P:VCC) IC60.14(P:VCC) IC61.14(P:VCC) IC62.14(P:VCC) IC63.14(P:VCC) IC64.14(P:VCC) IC65.14(P:VCC) IC66.14(P:VCC) IC67.14(P:VCC) IC68.14(P:VCC) IC69.14(P:VCC) IC70.14(P:VCC) IC71.14(P:VCC) IC73.14(P:VCC) IC74.5(VCC) IC75.5(VCC) IC76.14(P:VCC) IC77.14(P:VCC) IC78.14(P:VCC) IC81.14(P:VCC) IC82.14(P:VCC) IC83.14(P:VCC) IC84.14(P:VCC) IC85.14(P:VCC) IC86.14(P:VCC) IC87.14(P:VCC) IC88.14(VCC) IC89.14(P:VCC) IC90.14(P:VCC) IC91.14(P:VCC) IC92.14(P:VCC) IC93.14(P:VCC) IC94.14(P:VCC) IC95.14(P:VCC) IC96.14(P:VCC) IC97.14(P:VCC) IC98.14(P:VCC) IC99.14(P:VCC) IC100.14(P:VCC) IC101.5(VCC) IC102.5(VCC) IC103.5(VCC) IC104.14(P:VCC) IC105.14(P:VCC) IC106.5(VCC) IC107.5(VCC) IC108.14(P:VCC) IC109.14(P:VCC) IC110.14(P:VCC) IC111.14(P:VCC) U1.16(VCC) U2.16(VCC) U3.16(VCC) U4.16(VCC) U5.16(VCC) U6.16(VCC) U7.16(VCC) U8.16(VCC) U9.16(VCC) U10.16(VCC)

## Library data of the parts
C1 C2 = rcl:C-US: CAPACITOR, American symbol
C4-C7 = adafruit:C-US: CAPACITOR, American symbol
D1 D3-D5 = adafruit:1N4004: DIODE
FREIGHTERPROM1 FREIGHTERPROM2 IC39 IC41 IC43 IC79 = ic-package:DIL16: Dual In Line / Socket
IC1 IC17-IC19 IC23 IC27 IC30 IC45 IC49 IC61 IC66 IC67 IC92 IC100 IC111 = 74xx-us:74*04: Hex INVERTER
IC2 IC15 IC28 IC33 IC89 IC91 = 74xx-us:74*00: Quad 2-input NAND gate
IC3 IC11 IC32 IC93 = 74xx-us:74*107: Dual J-K FLIP FLOP, clear
IC4 IC5 IC9 IC10 = 74xx-us:74*93: Decade, divide by twelve and binary COUNTER
IC6 IC7 IC24 IC29 IC88 = 74xx-us:74*30: 8-input NAND gate
IC8 IC12 IC62 IC63 IC65 = 74xx-us:74*74: Dual D type positive edge triggered FLIP FLOP, preset and clear
IC13 IC16 IC84-IC86 IC98 = 74xx-us:74*10: Triple 3-input NAND gate
IC14 IC26 IC31 IC46 IC57 IC59 IC90 IC109 = 74xx-us:74*02: Quad 2-input NOR gate
IC20 = 74xx-us:74*86: Quad 2-input EXCLUSIV-OR (XOR) gate
IC21 IC25 IC34-IC36 IC42 IC48 IC51 IC58 IC64 IC78 IC81 IC82 IC94 IC99 IC104 IC105 IC108 IC110 = 74xx-us:74*08: Quad 2-input AND gate
IC22 IC37 IC38 IC52 IC53 IC60 IC68 IC69 IC77 IC83 IC95 IC97 = 74xx-us:74*32: Quad 2-input OR gate
IC40 IC54 IC87 = 74xx-us:74*27: Triple 3-input NOR gate
IC44 IC50 IC55 IC56 IC70 IC71 = 74xx-us:74*11: Triple 3-input AND gate
IC47 IC73 IC76 = 74xx-us:74*21: Dual 4-input AND gate
IC72 = SparkFun-IC-Special-Function:555: General purpose bipolar Timer Datasheet SparkFun Products SparkFun SparkPunk Sequencer Kit (KIT-12707) Storefront Component: 555 Timer (COM-09273) Two parts valid for production: VFP: IC-11930 (M7555 PTH) VFP: IC-09173 (555 PTH) - Preferred; PROD_ID: IC-09173; PROD_ID_ALT: IC-09173
IC74 IC75 IC101-IC103 IC106 IC107 = 74xx-us:74*90: Decade, divide by twelve and binary COUNTER
IC96 = 74xx-us:74*20: Dual 4-input NAND gate
Q1 = special:XTAL/S: CRYSTAL
Q2 = adafruit:2N2907*: PNP Transistor Big Oval pads
R1-R4 R6-R8 = rcl:R-US_: RESISTOR, American symbol
R5 R9-R41 R47 = adafruit:R-US_: RESISTOR, American symbol
SW1 SW2 = adafruit:SWITCH_PUSHBUTTON: Buttons
T1 T2 = adafruit:2N2222: NPN TRANSISTOR Big oval pads
U1-U10 = oldchips:74*161: Synchronous 4-bit COUNTER with direct clear
VR1 = SparkFun-Resistors:TRIMPOT: Trimming Potentiometer (Trimpot) Three-terminal potentiometers, with an adjustable wiper and two adjustable resistors. A pot can be used to create a configurable voltage divider, or as a variable resistor. "Trimpots" are a subset of potentiometers, usually intended for "set-and-forget"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; PROD_ID: RES-09730; SF_SKU: COM-09806; VALUE: 10k
X3 = con-sullinselectronics:050_610_?-22/44: .050 DIP EDGE CARD CONNECTOR .050 [1.27mm] CONTACT CENTERS .610" INSULATEOR HEIGHT Source: .050 DIP EDGE CARD.pdf; OC_FARNELL: unknown; OC_NEWARK: unknown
